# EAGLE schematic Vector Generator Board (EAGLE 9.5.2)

## Sheet 1 of 13: Power Supply & Negative Voltage generation
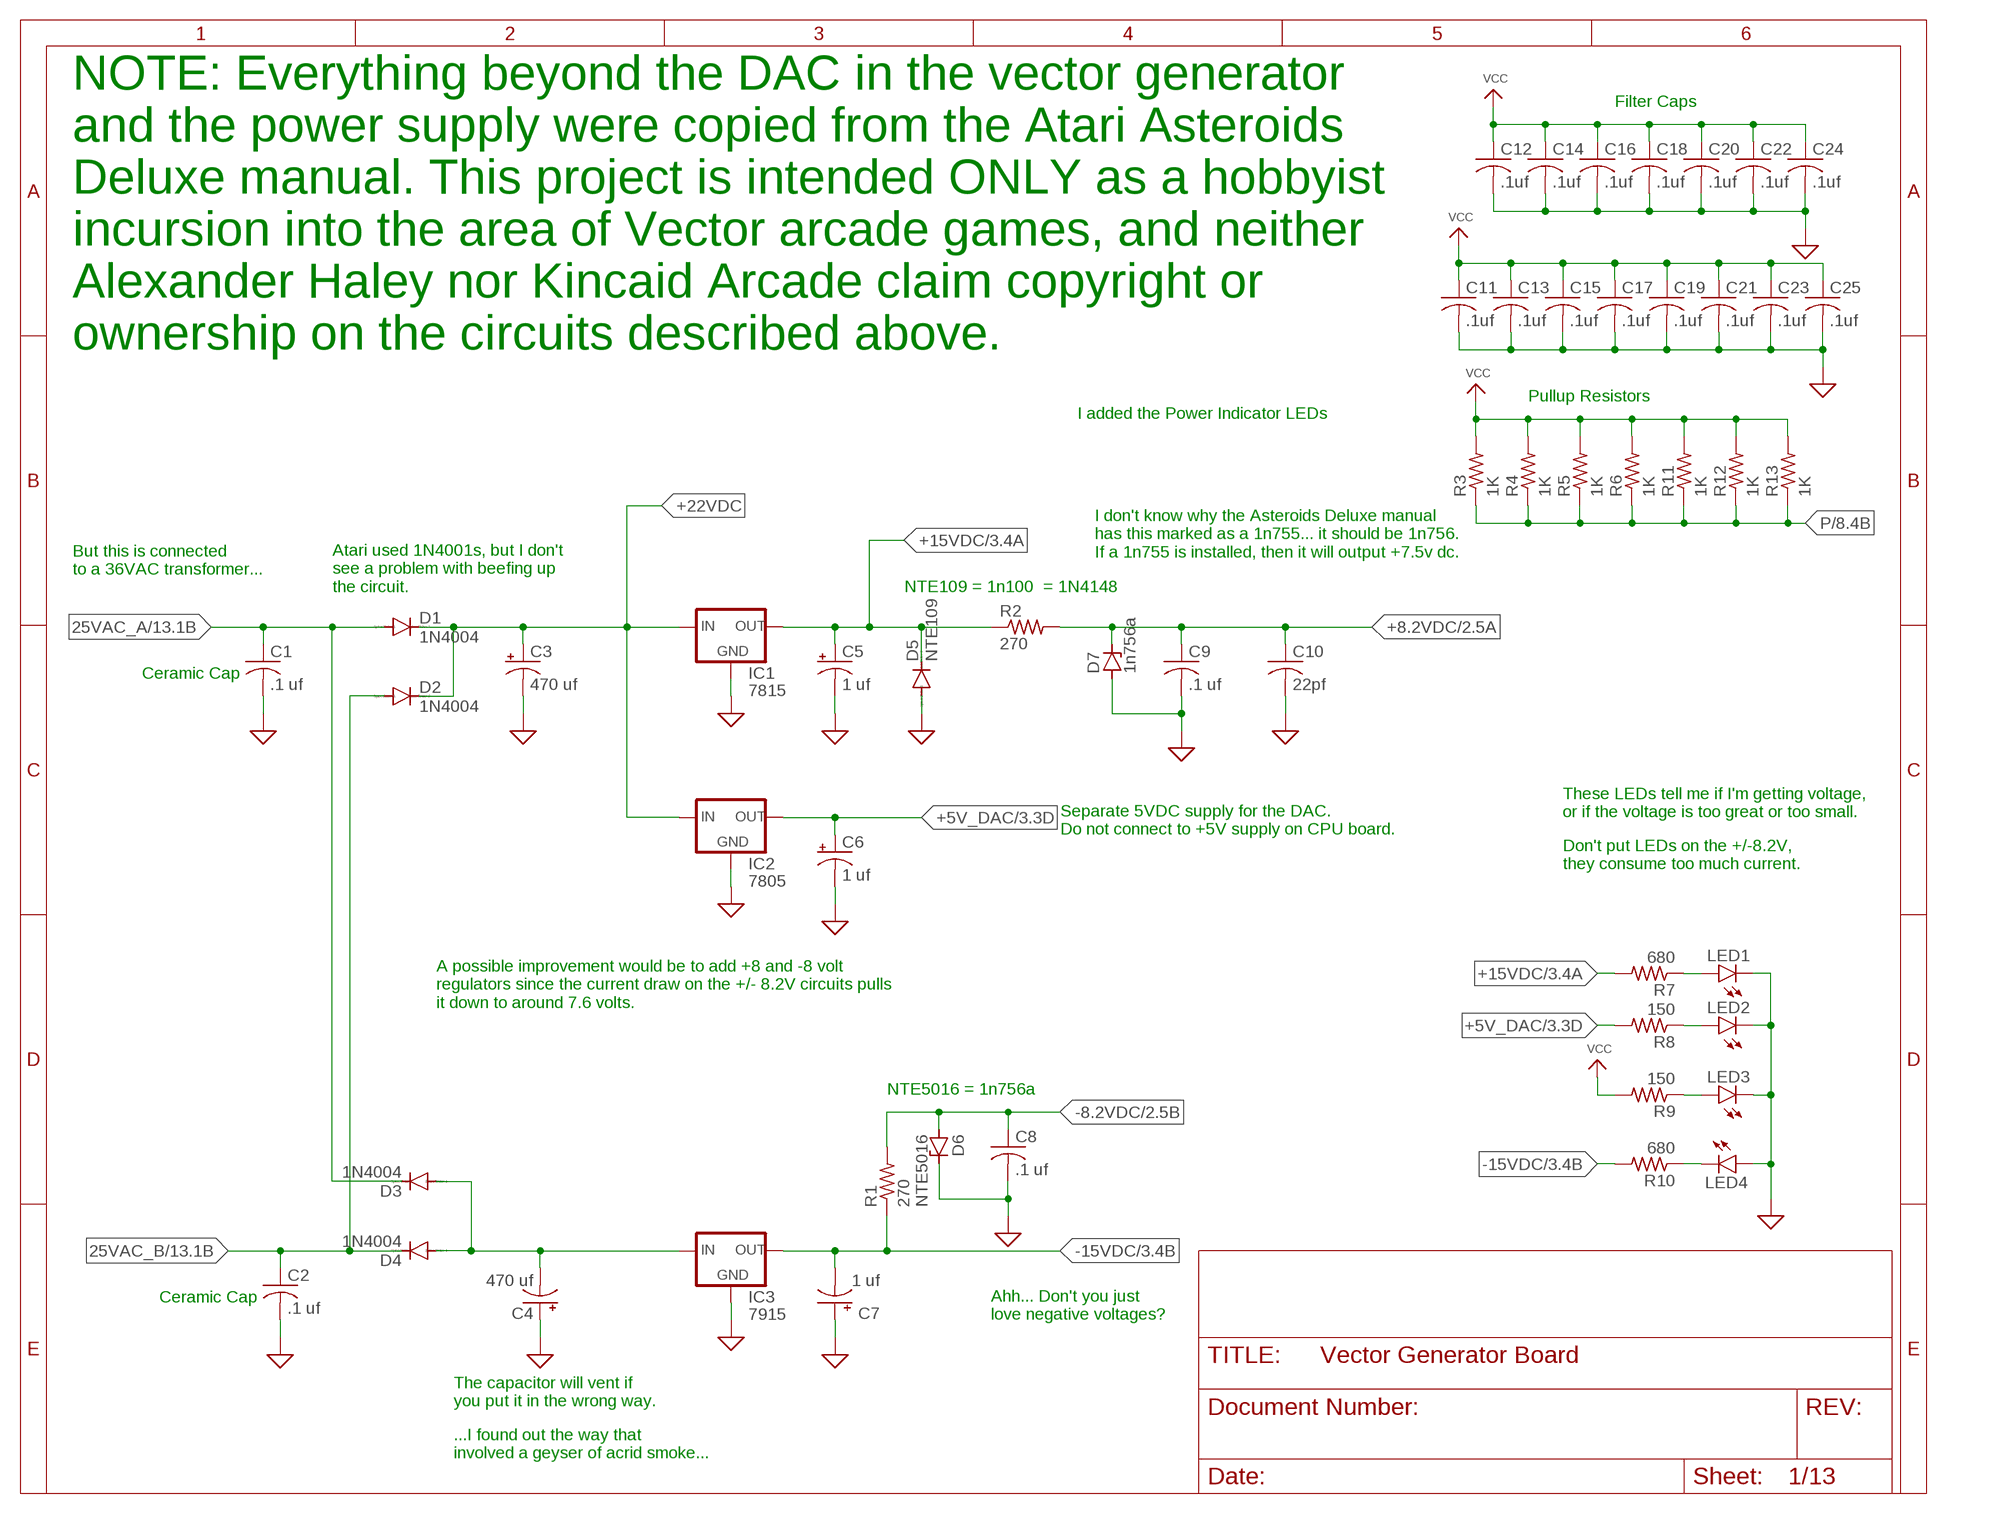
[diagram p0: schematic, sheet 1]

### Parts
C1  .1 uf  C-US050-050X075  [C050-050X075]
C2  .1 uf  C-US050-050X075  [C050-050X075]
C3  470 uf  CPOL-USE10-22.5  [EB22,5D]
C4  470 uf  CPOL-USE10-22.5  [EB22,5D]
C5  1 uf  CPOL-USB45181B  [B45181B]
C6  1 uf  CPOL-USB45181B  [B45181B]
C7  1 uf  CPOL-USB45181B  [B45181B]
C8  .1 uf  C-US050-050X075  [C050-050X075]
C9  .1 uf  C-US050-050X075  [C050-050X075]
C10  22pf  C-US050-050X075  [C050-050X075]
C11  .1uf  C-US050-030X075  [C050-030X075]
C12  .1uf  C-US050-030X075  [C050-030X075]
C13  .1uf  C-US050-030X075  [C050-030X075]
C14  .1uf  C-US050-030X075  [C050-030X075]
C15  .1uf  C-US050-030X075  [C050-030X075]
C16  .1uf  C-US050-030X075  [C050-030X075]
C17  .1uf  C-US050-030X075  [C050-030X075]
C18  .1uf  C-US050-030X075  [C050-030X075]
C19  .1uf  C-US050-030X075  [C050-030X075]
C20  .1uf  C-US050-030X075  [C050-030X075]
C21  .1uf  C-US050-030X075  [C050-030X075]
C22  .1uf  C-US050-030X075  [C050-030X075]
C23  .1uf  C-US050-030X075  [C050-030X075]
C24  .1uf  C-US050-030X075  [C050-030X075]
C25  .1uf  C-US050-030X075  [C050-030X075]
D1  1N4004  [DO41-10]
D2  1N4004  [DO41-10]
D3  1N4004  [DO41-10]
D4  1N4004  [DO41-10]
D5  NTE109  1N4004  [DO41-10]
D6  NTE5016  ZENER-DIODEDO35Z10  [DO35Z10]
D7  1n756a  ZENER-DIODEDO35Z10  [DO35Z10]
IC1  7815  78XXL  [78XXL]
IC2  7805  78XXL  [78XXL]
IC3  7915  78XXL  [78XXL]
LED1  LED3MM  [LED3MM]
LED2  LED3MM  [LED3MM]
LED3  LED3MM  [LED3MM]
LED4  LED3MM  [LED3MM]
R1  270  R-US_0207/12  [0207/12]
R2  270  R-US_0207/12  [0207/12]
R3  1K  R-US_0207/12  [0207/12]
R4  1K  R-US_0207/12  [0207/12]
R5  1K  R-US_0207/12  [0207/12]
R6  1K  R-US_0207/12  [0207/12]
R7  680  R-US_0207/12  [0207/12]
R8  150  R-US_0207/12  [0207/12]
R9  150  R-US_0207/12  [0207/12]
R10  680  R-US_0207/12  [0207/12]
R11  1K  R-US_0207/12  [0207/12]
R12  1K  R-US_0207/12  [0207/12]
R13  1K  R-US_0207/12  [0207/12]

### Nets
25VAC_A: C1.1 D1.A D3.C ; also sheet 13
25VAC_B: C2.1 D2.A D4.C ; also sheet 13
+5V_DAC: C6.+ IC2.OUT R8.2 ; also sheet 3,4
+8.2VDC: C9.1 C10.1 D7.C R2.2 ; also sheet 2,3,4,5
+15VDC: C5.+ D5.C IC1.OUT R2.1 R7.2 ; also sheet 3,4
+22VDC: C3.+ D1.C D2.C IC1.IN IC2.IN
-8.2VDC: C8.1 D6.A R1.2 ; also sheet 2,3,4,5
-15VDC: C7.- IC3.OUT R1.1 R10.2 ; also sheet 3,4
GND: C1.2 C2.2 C3.- C4.+ C5.- C6.- C7.+ C8.2 C9.2 C10.2 C11.2 C12.2 C13.2 C14.2 C15.2 C16.2 C17.2 C18.2 C19.2 C20.2 C21.2 C22.2 C23.2 C24.2 C25.2 D5.A D6.C D7.A IC1.GND IC2.GND IC3.GND LED1.K(C) LED2.K(C) LED3.K(C) LED4.A ; supply symbol labelled SUP ; also sheet 2,3,4,6,7,9,12,13
N$1: C4.- D3.A D4.A IC3.IN
N$6: LED1.A R7.1
N$8: LED2.A R8.1
N$9: LED3.A R9.1
N$123: LED4.K(C) R10.1
P: R3.1 R4.1 R5.1 R6.1 R11.1 R12.1 R13.1 ; also sheet 8,10,11,12
VCC: C11.1 C12.1 C13.1 C14.1 C15.1 C16.1 C17.1 C18.1 C19.1 C20.1 C21.1 C22.1 C23.1 C24.1 C25.1 R3.2 R4.2 R5.2 R6.2 R9.2 R11.2 R12.2 R13.2 ; also sheet 2,13

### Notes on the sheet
- Filter Caps
- NOTE: Everything beyond the DAC in the vector generator 
  and the power supply were copied from the Atari Asteroids 
  Deluxe manual. This project is intended ONLY as a hobbyist 
  incursion into the area of Vector arcade games, and neither 
  Alexander Haley nor Kincaid Arcade claim copyright or 
  ownership on the circuits described above.
- Pullup Resistors
- I added the Power Indicator LEDs
- I don't know why the Asteroids Deluxe manual
  has this marked as a 1n755... it should be 1n756.
  If a 1n755 is installed, then it will output +7.5v dc.
- But this is connected
  to a 36VAC transformer...
- Atari used 1N4001s, but I don't
  see a problem with beefing up
  the circuit.
- NTE109 = 1n100 | = 1N4148
- Ceramic Cap
- These LEDs tell me if I'm getting voltage,
  or if the voltage is too great or too small.
- Separate 5VDC supply for the DAC.
  Do not connect to +5V supply on CPU board.
- Don't put LEDs on the +/-8.2V,
  they consume too much current.
- A possible improvement would be to add +8 and -8 volt 
  regulators since the current draw on the +/- 8.2V circuits pulls 
  it down to around 7.6 volts.
- NTE5016 = 1n756a
- Ceramic Cap
- Ahh... Don't you just
  love negative voltages?
- The capacitor will vent if
  you put it in the wrong way.
- ...I found out the way that 
  involved a geyser of acrid smoke...

## Sheet 2 of 13: Z (Intensity) Out
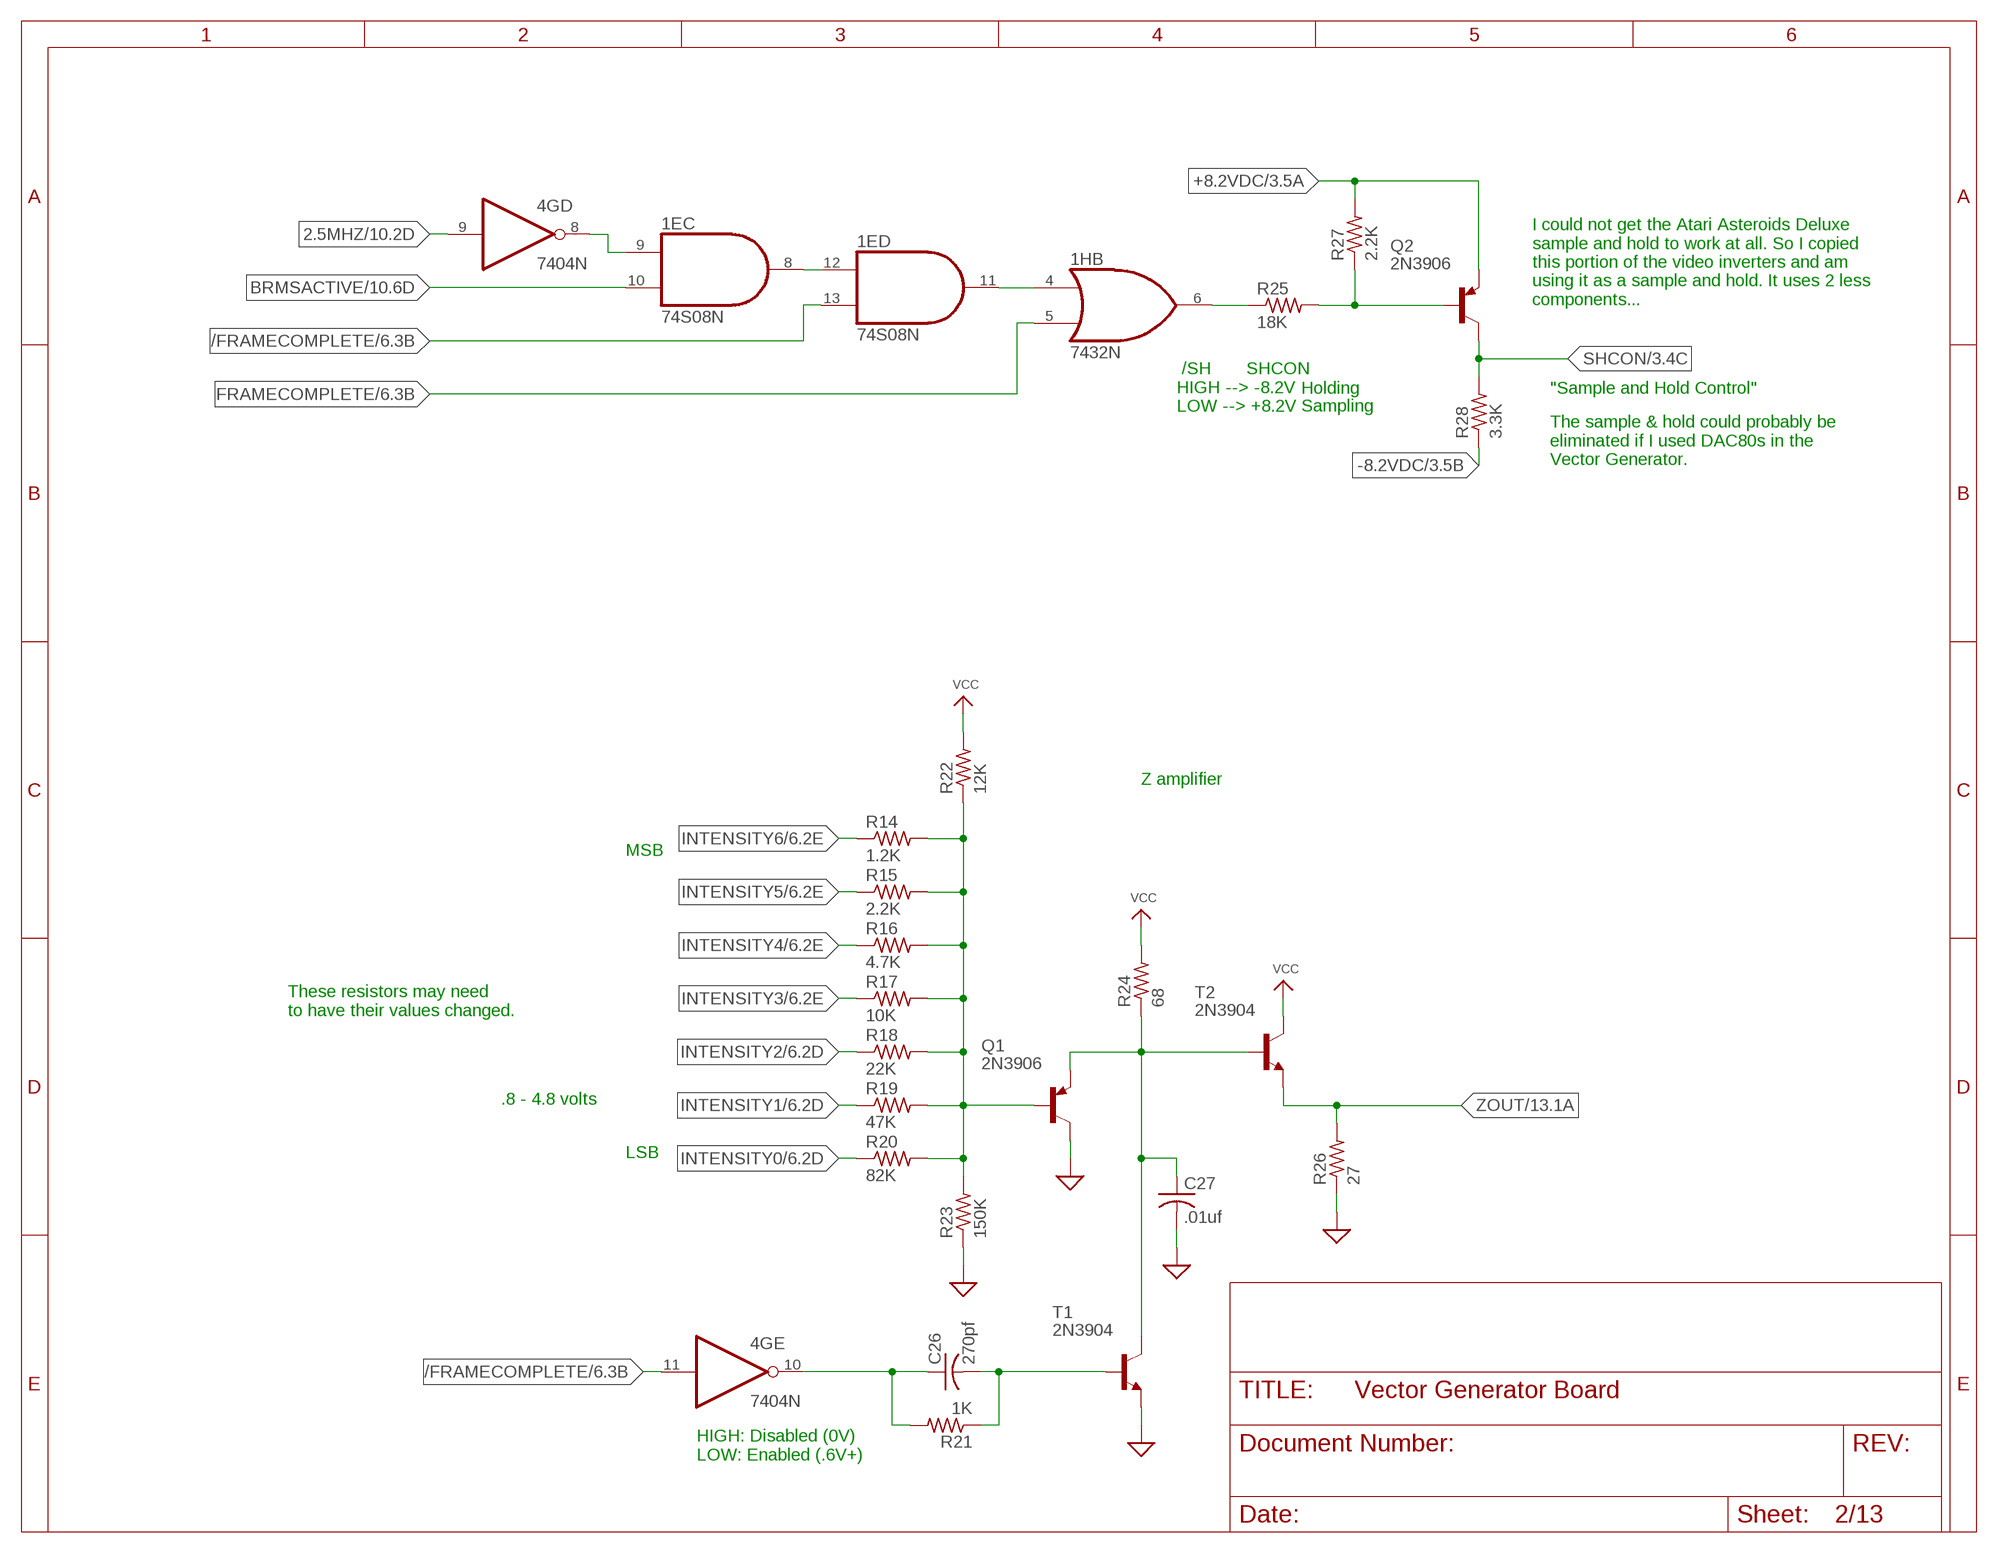
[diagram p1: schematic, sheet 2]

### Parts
1E  74S08N  [DIL14]
1H  7432N  [DIL14]
4G  7404N  [DIL14]
C26  270pf  C-US050-050X075  [C050-050X075]
C27  .01uf  C-US050-050X075  [C050-050X075]
Q1  2N3906  [TO92]
Q2  2N3906  [TO92]
R14  1.2K  R-US_0207/12  [0207/12]
R15  2.2K  R-US_0207/12  [0207/12]
R16  4.7K  R-US_0207/12  [0207/12]
R17  10K  R-US_0207/12  [0207/12]
R18  22K  R-US_0207/12  [0207/12]
R19  47K  R-US_0207/12  [0207/12]
R20  82K  R-US_0207/12  [0207/12]
R21  1K  R-US_0207/12  [0207/12]
R22  12K  R-US_0207/12  [0207/12]
R23  150K  R-US_0207/12  [0207/12]
R24  68  R-US_0207/12  [0207/12]
R25  18K  R-US_0207/12  [0207/12]
R26  27  R-US_0207/12  [0207/12]
R27  2.2K  R-US_0207/12  [0207/12]
R28  3.3K  R-US_0207/12  [0207/12]
T1  2N3904  [TO92]
T2  2N3904  [TO92]

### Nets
2.5MHZ: 4G.9(D:I) ; also sheet 10,13
+8.2VDC: Q2.3(E) R27.2 ; also sheet 1,3,4,5
-8.2VDC: R28.1 ; also sheet 1,3,4,5
/FRAMECOMPLETE: 1E.13(D:I1) 4G.11(E:I) ; also sheet 6
BRMSACTIVE: 1E.10(C:I1) ; also sheet 10
FRAMECOMPLETE: 1H.5(B:I1) ; also sheet 6,13
GND: C27.2 Q1.1(C) R23.1 R26.1 T1.3(E) ; supply symbol labelled SUP ; also sheet 1,3,4,6,7,9,12,13
INTENSITY0: R20.1 ; also sheet 6,11
INTENSITY1: R19.1 ; also sheet 6,11
INTENSITY2: R18.1 ; also sheet 6,11
INTENSITY3: R17.1 ; also sheet 6,11
INTENSITY4: R16.1 ; also sheet 6,11
INTENSITY5: R15.1 ; also sheet 6,11
INTENSITY6: R14.1 ; also sheet 6,11
N$2: 1H.6(B:O) R25.1
N$3: 1E.11(D:O) 1H.4(B:I0)
N$4: Q1.2(B) R14.2 R15.2 R16.2 R17.2 R18.2 R19.2 R20.2 R22.1 R23.2
N$5: Q2.2(B) R25.2 R27.1
N$12: C27.1 Q1.3(E) R24.1 T1.1(C) T2.2(B)
N$14: C26.2 R21.1 T1.2(B)
N$15: 4G.10(E:O) C26.1 R21.2
N$46: 1E.8(C:O) 1E.12(D:I0)
N$100: 1E.9(C:I0) 4G.8(D:O)
SHCON: Q2.1(C) R28.2 ; also sheet 3,4
VCC: R22.2 R24.2 T2.1(C) ; also sheet 1,13
ZOUT: R26.2 T2.3(E) ; also sheet 13

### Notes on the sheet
- I could not get the Atari Asteroids Deluxe
  sample and hold to work at all. So I copied
  this portion of the video inverters and am
  using it as a sample and hold. It uses 2 less
  components...
- Holding | "Sample and Hold Control"
- /SH       SHCON
  HIGH --> -8.2V
  LOW --> +8.2V
- Sampling
- The sample & hold could probably be 
  eliminated if I used DAC80s in the 
  Vector Generator.
- Z amplifier
- MSB
- These resistors may need 
  to have their values changed.
- .8 - 4.8 volts
- LSB
- HIGH: Disabled (0V)
  LOW: Enabled (.6V+)

## Sheet 3 of 13: X Out
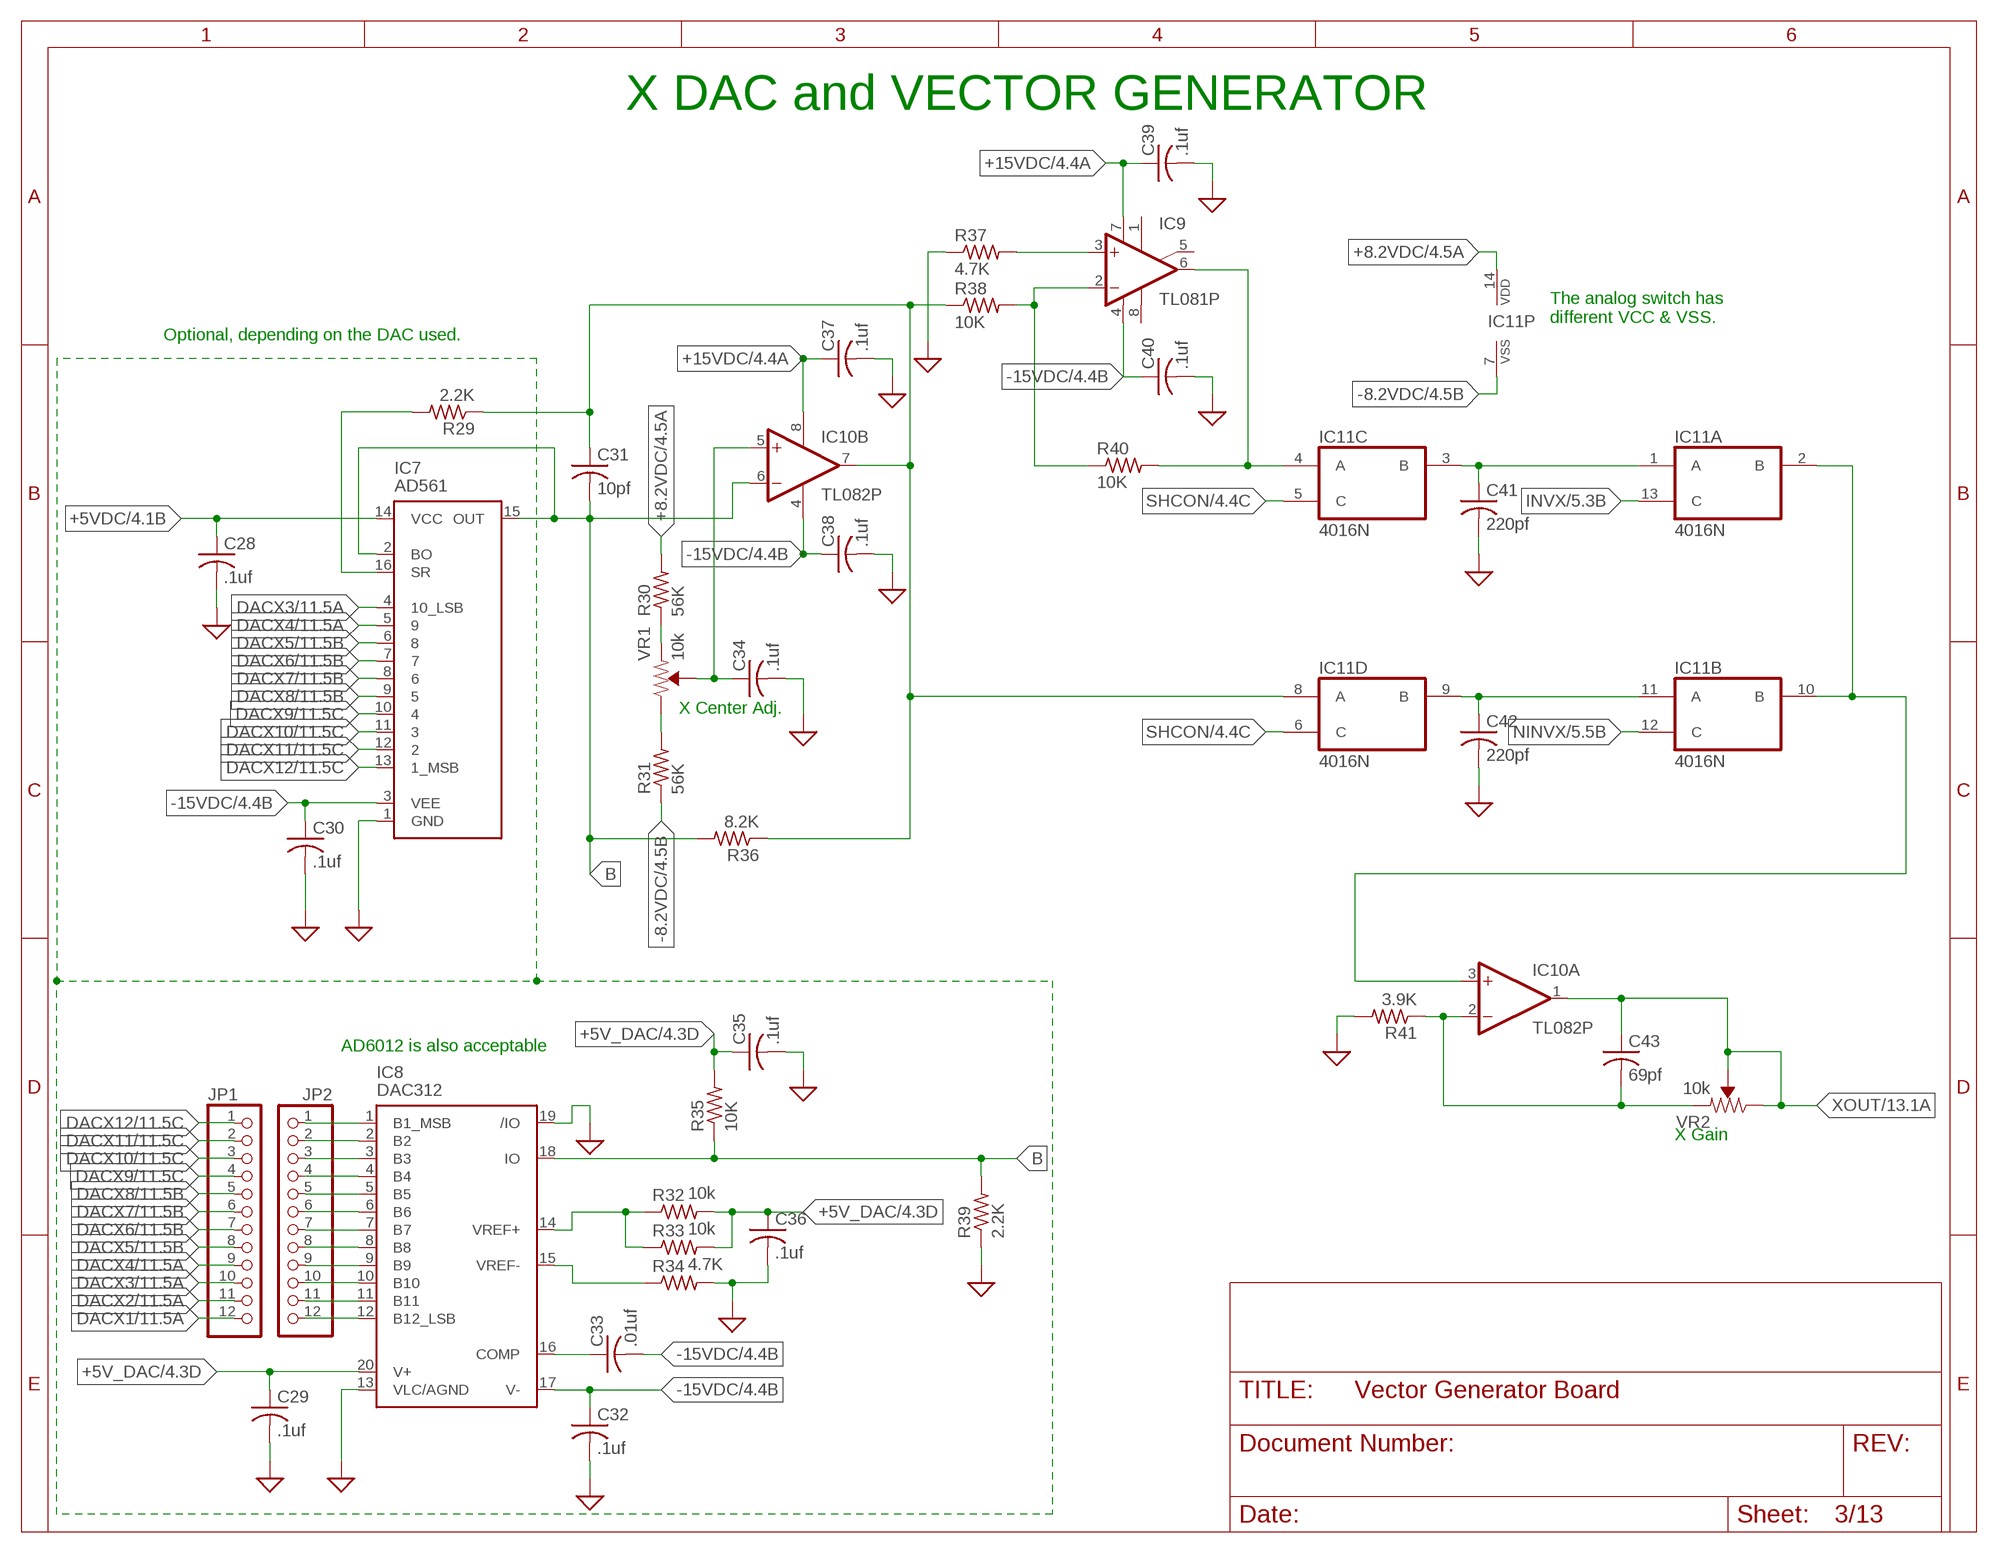
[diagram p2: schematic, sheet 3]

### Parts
C28  .1uf  C-US050-050X075  [C050-050X075]
C29  .1uf  C-US050-050X075  [C050-050X075]
C30  .1uf  C-US050-050X075  [C050-050X075]
C31  10pf  C-US050-050X075  [C050-050X075]
C32  .1uf  C-US050-050X075  [C050-050X075]
C33  .01uf  C-US050-050X075  [C050-050X075]
C34  .1uf  C-US050-050X075  [C050-050X075]
C35  .1uf  C-US050-050X075  [C050-050X075]
C36  .1uf  C-US050-050X075  [C050-050X075]
C37  .1uf  C-US050-050X075  [C050-050X075]
C38  .1uf  C-US050-050X075  [C050-050X075]
C39  .1uf  C-US050-050X075  [C050-050X075]
C40  .1uf  C-US050-050X075  [C050-050X075]
C41  220pf  C-US050-050X075  [C050-050X075]
C42  220pf  C-US050-050X075  [C050-050X075]
C43  69pf  C-US050-050X075  [C050-050X075]
IC7  AD561  [DIL16]
IC8  DAC312  [DIL20]
IC9  TL081P  [DIL08]
IC10  TL082P  [DIL08]
IC11  4016N  [DIL14]
JP1  PINHD-1X12  [1X12]
JP2  PINHD-1X12  [1X12]
R29  2.2K  R-US_0207/12  [0207/12]
R30  56K  R-US_0207/12  [0207/12]
R31  56K  R-US_0207/12  [0207/12]
R32  10k  R-US_0207/12  [0207/12]
R33  10k  R-US_0207/12  [0207/12]
R34  4.7K  R-US_0207/12  [0207/12]
R35  10K  R-US_0207/12  [0207/12]
R36  8.2K  R-US_0207/12  [0207/12]
R37  4.7K  R-US_0207/12  [0207/12]
R38  10K  R-US_0207/12  [0207/12]
R39  2.2K  R-US_0207/12  [0207/12]
R40  10K  R-US_0207/12  [0207/12]
R41  3.9K  R-US_0207/12  [0207/12]
VR1  10k  TRIMPOT-PTH-10MM-KNOB-1/2W-10%  [TRIMPOT-PTH-3386U]
VR2  10k  TRIMPOT-PTH-10MM-KNOB-1/2W-10%  [TRIMPOT-PTH-3386U]

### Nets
+5V_DAC: C29.1 C35.1 C36.1 IC8.20(V+) R32.2 R33.2 R35.2 ; also sheet 1,4
+5VDC: C28.1 IC7.14(VCC) ; also sheet 4
+8.2VDC: IC11.14(P:VDD) R30.2 ; also sheet 1,2,4,5
+15VDC: C37.1 C39.1 IC9.7(V+) IC10.8(P:V+) ; also sheet 1,4
-8.2VDC: IC11.7(P:VSS) R31.1 ; also sheet 1,2,4,5
-15VDC: C30.1 C32.1 C33.2 C38.1 C40.1 IC7.3(VEE) IC8.17(V-) IC9.4(V-) IC10.4(P:V-) ; also sheet 1,4
B: C31.2 IC7.2(BO) IC7.15(OUT) IC8.18(IO) IC10.6(B:-IN) R35.1 R36.2 R39.2
DACX1: JP1.12 ; also sheet 11,12
DACX2: JP1.11 ; also sheet 11,12
DACX3: IC7.4(10_LSB) JP1.10 ; also sheet 11,12
DACX4: IC7.5 JP1.9 ; also sheet 11,12
DACX5: IC7.6 JP1.8 ; also sheet 11,12
DACX6: IC7.7 JP1.7 ; also sheet 11,12
DACX7: IC7.8 JP1.6 ; also sheet 11,12
DACX8: IC7.9 JP1.5 ; also sheet 11,12
DACX9: IC7.10 JP1.4 ; also sheet 11,12
DACX10: IC7.11 JP1.3 ; also sheet 11,12
DACX11: IC7.12 JP1.2 ; also sheet 11,12
DACX12: IC7.13(1_MSB) JP1.1 ; also sheet 11,12
GND: C28.2 C29.2 C30.2 C32.2 C34.2 C35.2 C36.2 C37.2 C38.2 C39.2 C40.2 C41.2 C42.2 IC7.1(GND) IC8.13(VLC/AGND) IC8.19(/IO) R34.2 R37.1 R39.1 R41.2 ; supply symbol labelled SUP ; also sheet 1,2,4,6,7,9,12,13
INVX: IC11.13(A:C) ; also sheet 5
N$11: C31.1 IC10.7(B:OUT) IC11.8(D:A) R29.1 R36.1 R38.1
N$13: IC7.16(SR) R29.2
N$16: C41.1 IC11.1(A:A) IC11.3(C:B)
N$17: C42.1 IC11.9(D:B) IC11.11(B:A)
N$18: IC10.3(A:+IN) IC11.2(A:B) IC11.10(B:B)
N$19: IC9.2(-IN) R38.2 R40.1
N$20: IC9.3(+IN) R37.2
N$21: IC9.6(OUT) IC11.4(C:A) R40.2
N$23: C43.2 IC10.2(A:-IN) R41.1 VR2.1(CCW)
N$57: R31.2 VR1.3(CW)
N$108: IC8.1(B1_MSB) JP2.1
N$109: IC8.2(B2) JP2.2
N$110: IC8.3(B3) JP2.3
N$119: R30.1 VR1.1(CCW)
N$120: C33.1 IC8.16(COMP)
N$121: IC8.14(VREF+) R32.1 R33.1
N$122: IC8.15(VREF-) R34.1
N$124: C34.1 IC10.5(B:+IN) VR1.2(WIPER)
N$125: IC8.4(B4) JP2.4
N$128: IC8.5(B5) JP2.5
N$130: IC8.6(B6) JP2.6
N$131: IC8.7(B7) JP2.7
N$132: IC8.8(B8) JP2.8
N$133: IC8.9(B9) JP2.9
N$134: IC8.10(B10) JP2.10
N$135: IC8.11(B11) JP2.11
N$136: IC8.12(B12_LSB) JP2.12
NINVX: IC11.12(B:C) ; also sheet 5
SHCON: IC11.5(C:C) IC11.6(D:C) ; also sheet 2,4
XOUT: C43.1 IC10.1(A:OUT) VR2.2(WIPER) VR2.3(CW) ; also sheet 13
Unconnected: IC9.1(ON1) IC9.5(ON2) IC9.8(OPT)

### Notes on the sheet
- X DAC and VECTOR GENERATOR
- The analog switch has
  different VCC & VSS.
- Optional, depending on the DAC used.
- X Center Adj.
- AD6012 is also acceptable
- X Gain

## Sheet 4 of 13: Y Out
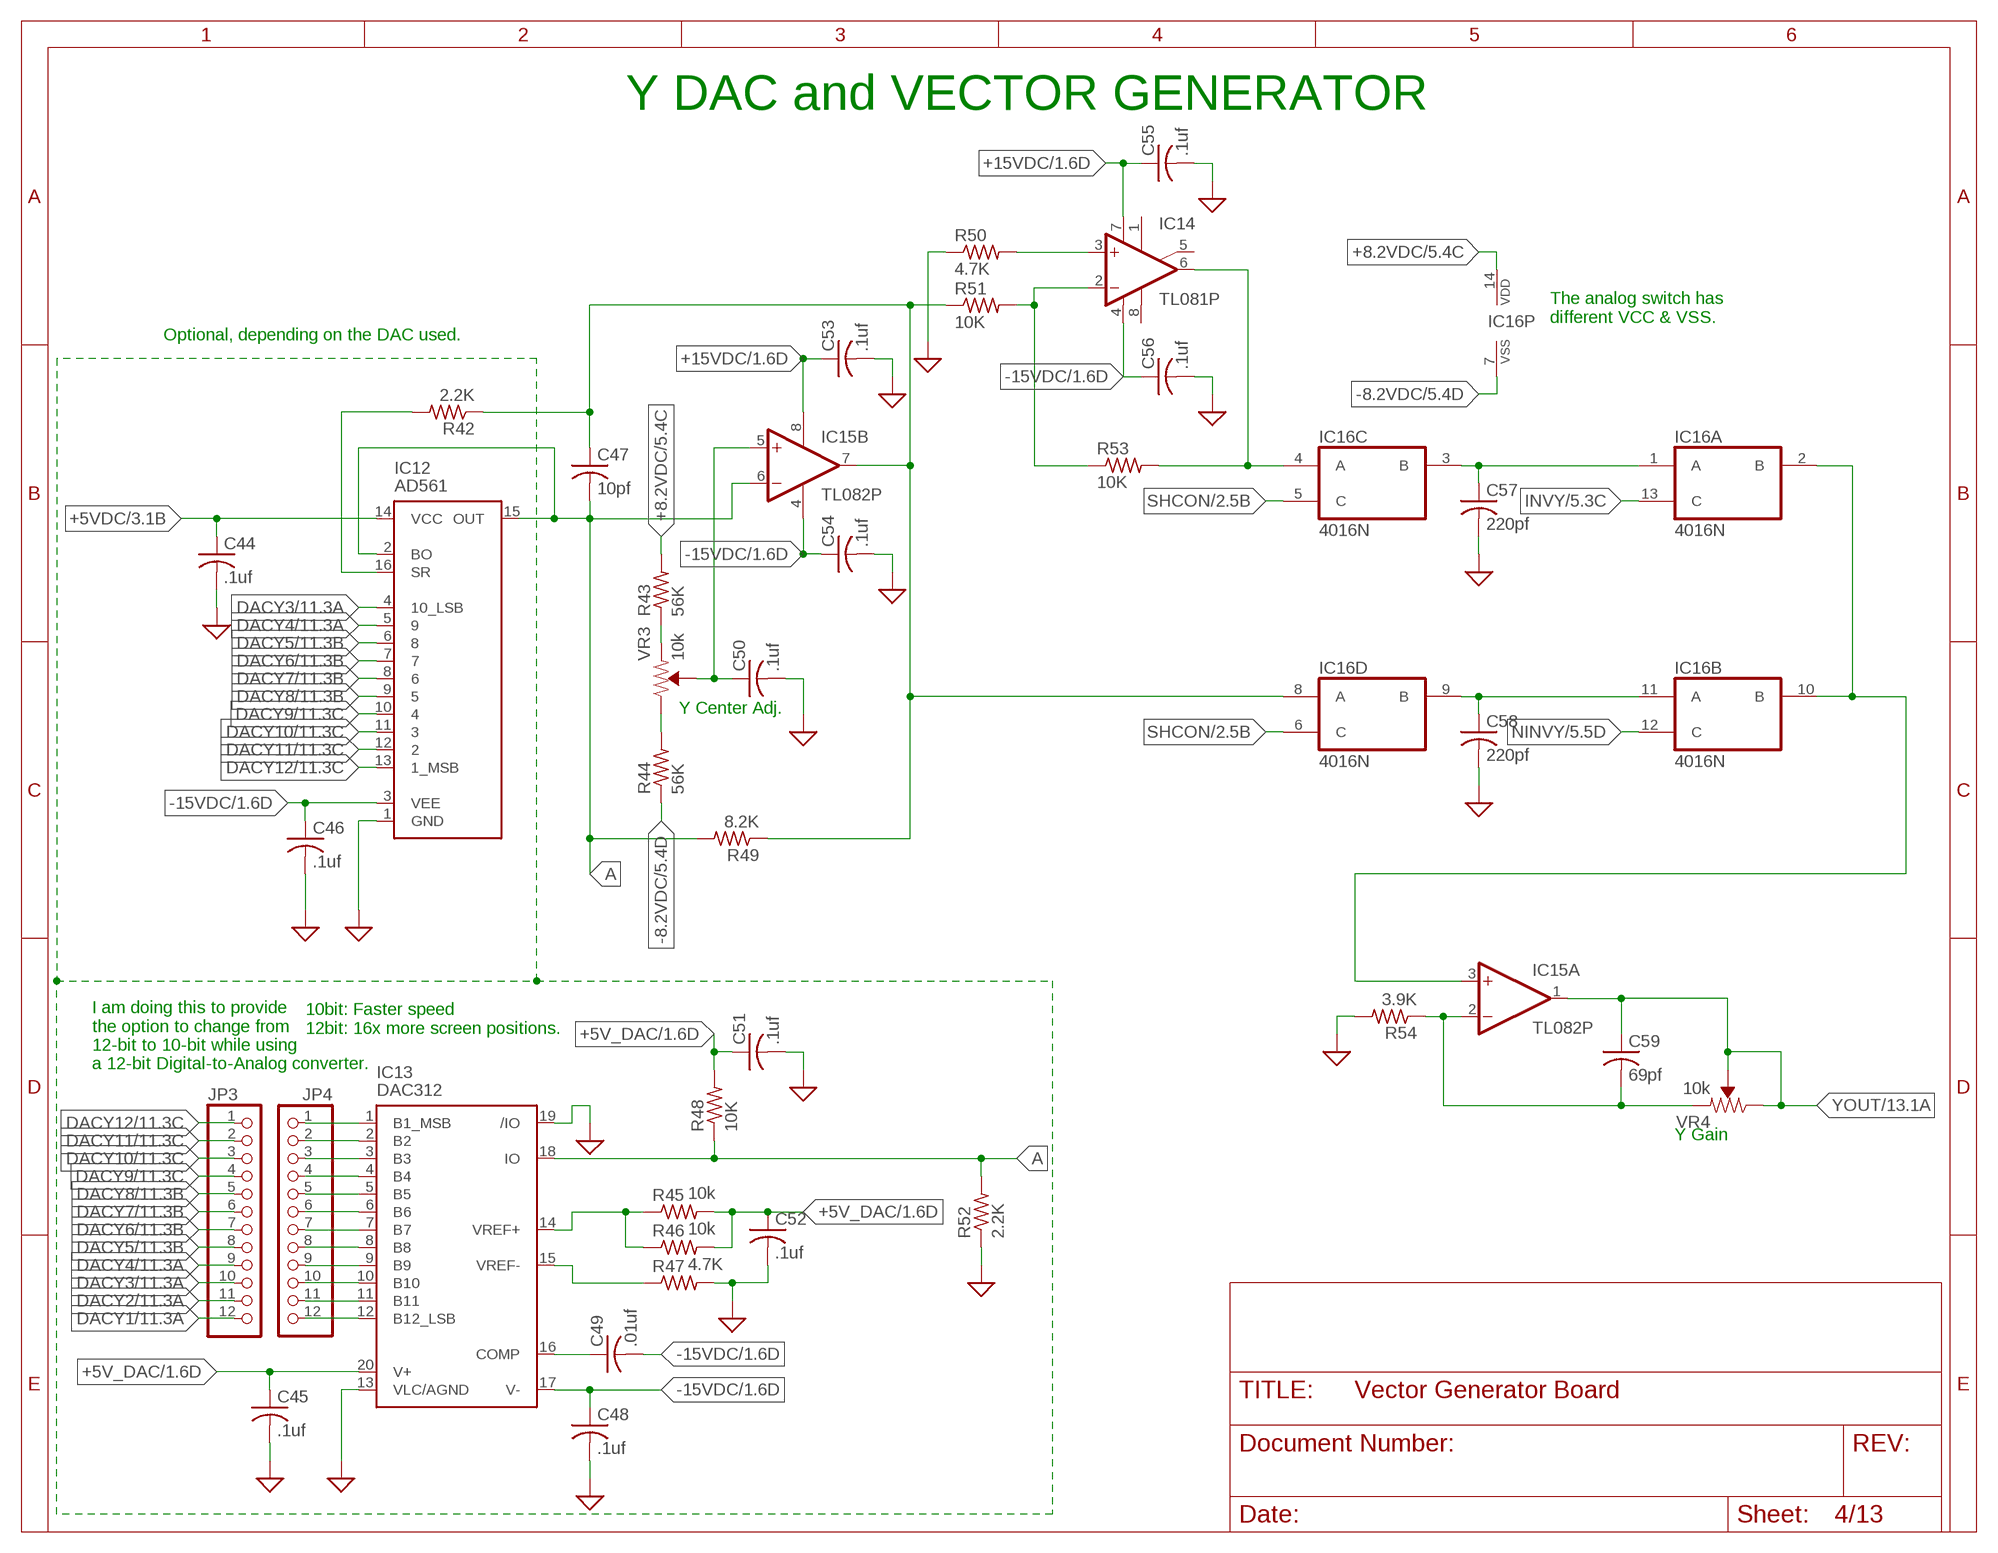
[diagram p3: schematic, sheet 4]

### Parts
C44  .1uf  C-US050-050X075  [C050-050X075]
C45  .1uf  C-US050-050X075  [C050-050X075]
C46  .1uf  C-US050-050X075  [C050-050X075]
C47  10pf  C-US050-050X075  [C050-050X075]
C48  .1uf  C-US050-050X075  [C050-050X075]
C49  .01uf  C-US050-050X075  [C050-050X075]
C50  .1uf  C-US050-050X075  [C050-050X075]
C51  .1uf  C-US050-050X075  [C050-050X075]
C52  .1uf  C-US050-050X075  [C050-050X075]
C53  .1uf  C-US050-050X075  [C050-050X075]
C54  .1uf  C-US050-050X075  [C050-050X075]
C55  .1uf  C-US050-050X075  [C050-050X075]
C56  .1uf  C-US050-050X075  [C050-050X075]
C57  220pf  C-US050-050X075  [C050-050X075]
C58  220pf  C-US050-050X075  [C050-050X075]
C59  69pf  C-US050-050X075  [C050-050X075]
IC12  AD561  [DIL16]
IC13  DAC312  [DIL20]
IC14  TL081P  [DIL08]
IC15  TL082P  [DIL08]
IC16  4016N  [DIL14]
JP3  PINHD-1X12  [1X12]
JP4  PINHD-1X12  [1X12]
R42  2.2K  R-US_0207/12  [0207/12]
R43  56K  R-US_0207/12  [0207/12]
R44  56K  R-US_0207/12  [0207/12]
R45  10k  R-US_0207/12  [0207/12]
R46  10k  R-US_0207/12  [0207/12]
R47  4.7K  R-US_0207/12  [0207/12]
R48  10K  R-US_0207/12  [0207/12]
R49  8.2K  R-US_0207/12  [0207/12]
R50  4.7K  R-US_0207/12  [0207/12]
R51  10K  R-US_0207/12  [0207/12]
R52  2.2K  R-US_0207/12  [0207/12]
R53  10K  R-US_0207/12  [0207/12]
R54  3.9K  R-US_0207/12  [0207/12]
VR3  10k  TRIMPOT-PTH-10MM-KNOB-1/2W-10%  [TRIMPOT-PTH-3386U]
VR4  10k  TRIMPOT-PTH-10MM-KNOB-1/2W-10%  [TRIMPOT-PTH-3386U]

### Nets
+5V_DAC: C45.1 C51.1 C52.1 IC13.20(V+) R45.2 R46.2 R48.2 ; also sheet 1,3
+5VDC: C44.1 IC12.14(VCC) ; also sheet 3
+8.2VDC: IC16.14(P:VDD) R43.2 ; also sheet 1,2,3,5
+15VDC: C53.1 C55.1 IC14.7(V+) IC15.8(P:V+) ; also sheet 1,3
-8.2VDC: IC16.7(P:VSS) R44.1 ; also sheet 1,2,3,5
-15VDC: C46.1 C48.1 C49.2 C54.1 C56.1 IC12.3(VEE) IC13.17(V-) IC14.4(V-) IC15.4(P:V-) ; also sheet 1,3
A: C47.2 IC12.2(BO) IC12.15(OUT) IC13.18(IO) IC15.6(B:-IN) R48.1 R49.2 R52.2
DACY1: JP3.12 ; also sheet 11,12
DACY2: JP3.11 ; also sheet 11,12
DACY3: IC12.4(10_LSB) JP3.10 ; also sheet 11,12
DACY4: IC12.5 JP3.9 ; also sheet 11,12
DACY5: IC12.6 JP3.8 ; also sheet 11,12
DACY6: IC12.7 JP3.7 ; also sheet 11,12
DACY7: IC12.8 JP3.6 ; also sheet 11,12
DACY8: IC12.9 JP3.5 ; also sheet 11,12
DACY9: IC12.10 JP3.4 ; also sheet 11,12
DACY10: IC12.11 JP3.3 ; also sheet 11,12
DACY11: IC12.12 JP3.2 ; also sheet 11,12
DACY12: IC12.13(1_MSB) JP3.1 ; also sheet 11,12
GND: C44.2 C45.2 C46.2 C48.2 C50.2 C51.2 C52.2 C53.2 C54.2 C55.2 C56.2 C57.2 C58.2 IC12.1(GND) IC13.13(VLC/AGND) IC13.19(/IO) R47.2 R50.1 R52.1 R54.2 ; supply symbol labelled SUP ; also sheet 1,2,3,6,7,9,12,13
INVY: IC16.13(A:C) ; also sheet 5
N$10: R44.2 VR3.3(CW)
N$22: IC13.1(B1_MSB) JP4.1
N$24: IC13.2(B2) JP4.2
N$25: C47.1 IC15.7(B:OUT) IC16.8(D:A) R42.1 R49.1 R51.1
N$26: IC12.16(SR) R42.2
N$27: C57.1 IC16.1(A:A) IC16.3(C:B)
N$28: C58.1 IC16.9(D:B) IC16.11(B:A)
N$29: IC15.3(A:+IN) IC16.2(A:B) IC16.10(B:B)
N$30: IC14.2(-IN) R51.2 R53.1
N$31: IC14.3(+IN) R50.2
N$32: IC14.6(OUT) IC16.4(C:A) R53.2
N$33: C59.2 IC15.2(A:-IN) R54.1 VR4.1(CCW)
N$44: IC13.3(B3) JP4.3
N$45: IC13.4(B4) JP4.4
N$54: IC13.5(B5) JP4.5
N$55: IC13.6(B6) JP4.6
N$56: IC13.7(B7) JP4.7
N$71: IC13.8(B8) JP4.8
N$98: IC13.9(B9) JP4.9
N$105: IC13.10(B10) JP4.10
N$106: IC13.11(B11) JP4.11
N$107: IC13.12(B12_LSB) JP4.12
N$115: IC13.14(VREF+) R45.1 R46.1
N$116: C49.1 IC13.16(COMP)
N$118: IC13.15(VREF-) R47.1
N$126: R43.1 VR3.1(CCW)
N$127: C50.1 IC15.5(B:+IN) VR3.2(WIPER)
NINVY: IC16.12(B:C) ; also sheet 5
SHCON: IC16.5(C:C) IC16.6(D:C) ; also sheet 2,3
YOUT: C59.1 IC15.1(A:OUT) VR4.2(WIPER) VR4.3(CW) ; also sheet 13
Unconnected: IC14.1(ON1) IC14.5(ON2) IC14.8(OPT)

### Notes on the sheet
- Y DAC and VECTOR GENERATOR
- The analog switch has
  different VCC & VSS.
- Optional, depending on the DAC used.
- Y Center Adj.
- 10bit: Faster speed
  12bit: 16x more screen positions.
- I am doing this to provide
  the option to change from
  12-bit to 10-bit while using
  a 12-bit Digital-to-Analog converter.
- Y Gain

## Sheet 5 of 13: Video Inverter
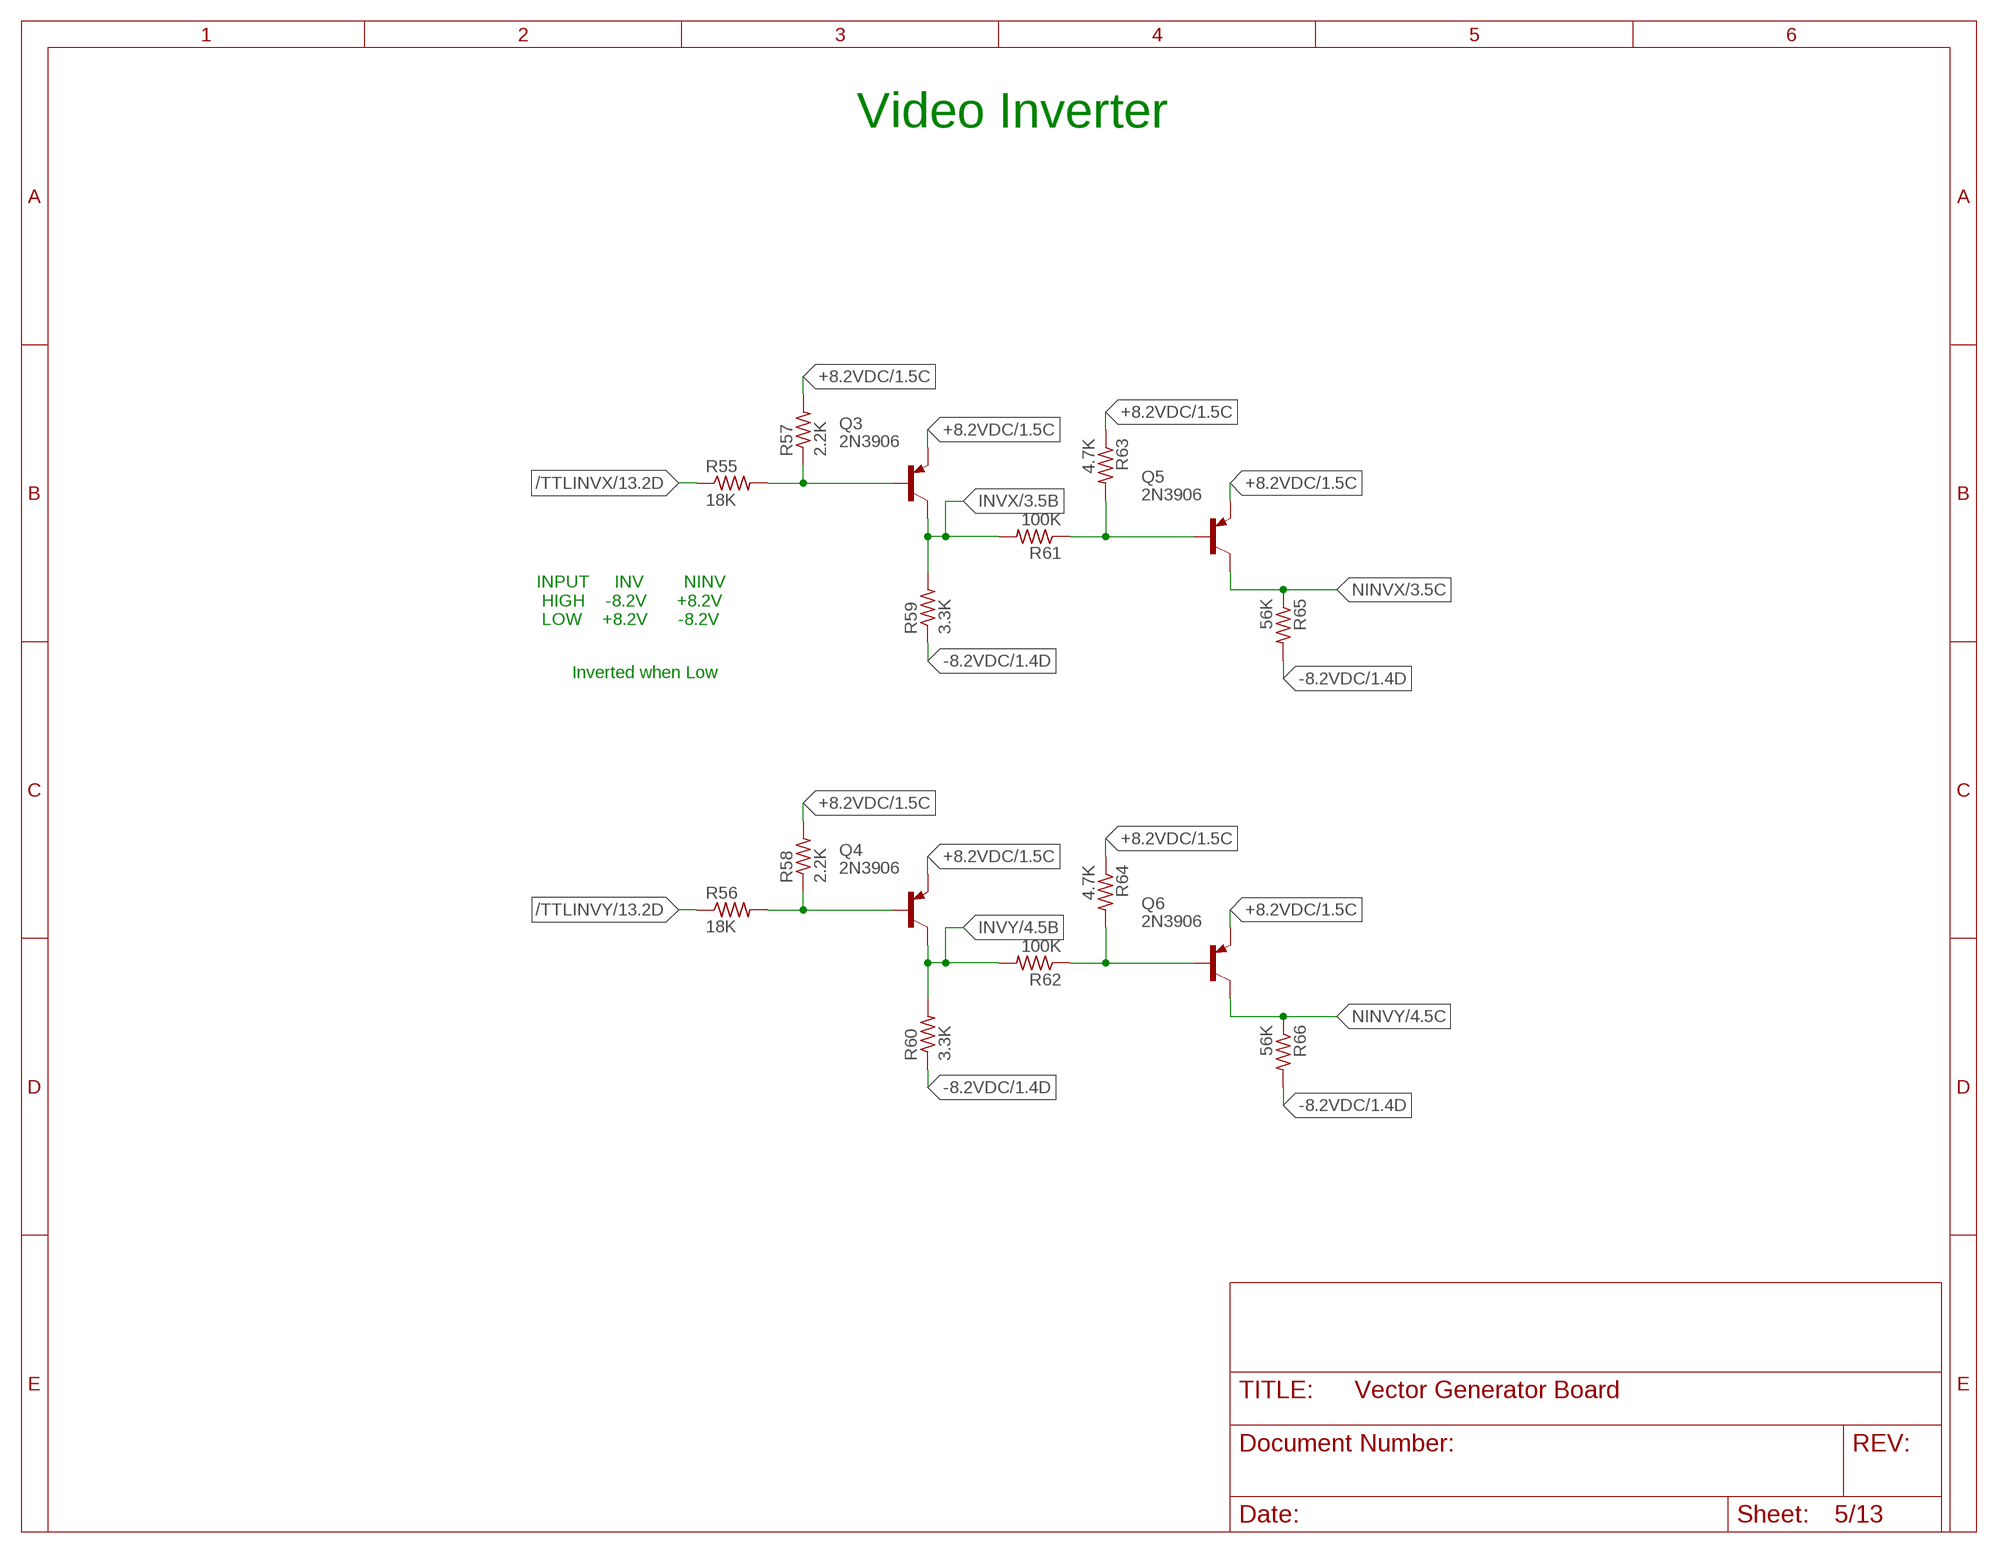
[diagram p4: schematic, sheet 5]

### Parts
Q3  2N3906  [TO92]
Q4  2N3906  [TO92]
Q5  2N3906  [TO92]
Q6  2N3906  [TO92]
R55  18K  R-US_0207/12  [0207/12]
R56  18K  R-US_0207/12  [0207/12]
R57  2.2K  R-US_0207/12  [0207/12]
R58  2.2K  R-US_0207/12  [0207/12]
R59  3.3K  R-US_0207/12  [0207/12]
R60  3.3K  R-US_0207/12  [0207/12]
R61  100K  R-US_0207/12  [0207/12]
R62  100K  R-US_0207/12  [0207/12]
R63  4.7K  R-US_0207/12  [0207/12]
R64  4.7K  R-US_0207/12  [0207/12]
R65  56K  R-US_0207/12  [0207/12]
R66  56K  R-US_0207/12  [0207/12]

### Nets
+8.2VDC: Q3.3(E) Q4.3(E) Q5.3(E) Q6.3(E) R57.2 R58.2 R63.1 R64.1 ; also sheet 1,2,3,4
-8.2VDC: R59.1 R60.1 R65.2 R66.2 ; also sheet 1,2,3,4
/TTLINVX: R55.1 ; also sheet 13
/TTLINVY: R56.1 ; also sheet 13
INVX: Q3.1(C) R59.2 R61.2 ; also sheet 3
INVY: Q4.1(C) R60.2 R62.2 ; also sheet 4
N$35: Q3.2(B) R55.2 R57.1
N$37: Q4.2(B) R56.2 R58.1
N$38: Q6.2(B) R62.1 R64.2
N$39: Q5.2(B) R61.1 R63.2
NINVX: Q5.1(C) R65.1 ; also sheet 3
NINVY: Q6.1(C) R66.1 ; also sheet 4

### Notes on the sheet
- Video Inverter
- INPUT     INV        NINV
   HIGH    -8.2V      +8.2V
   LOW    +8.2V      -8.2V
- Inverted when Low

## Sheet 6 of 13: Input Latches & Stage Counter
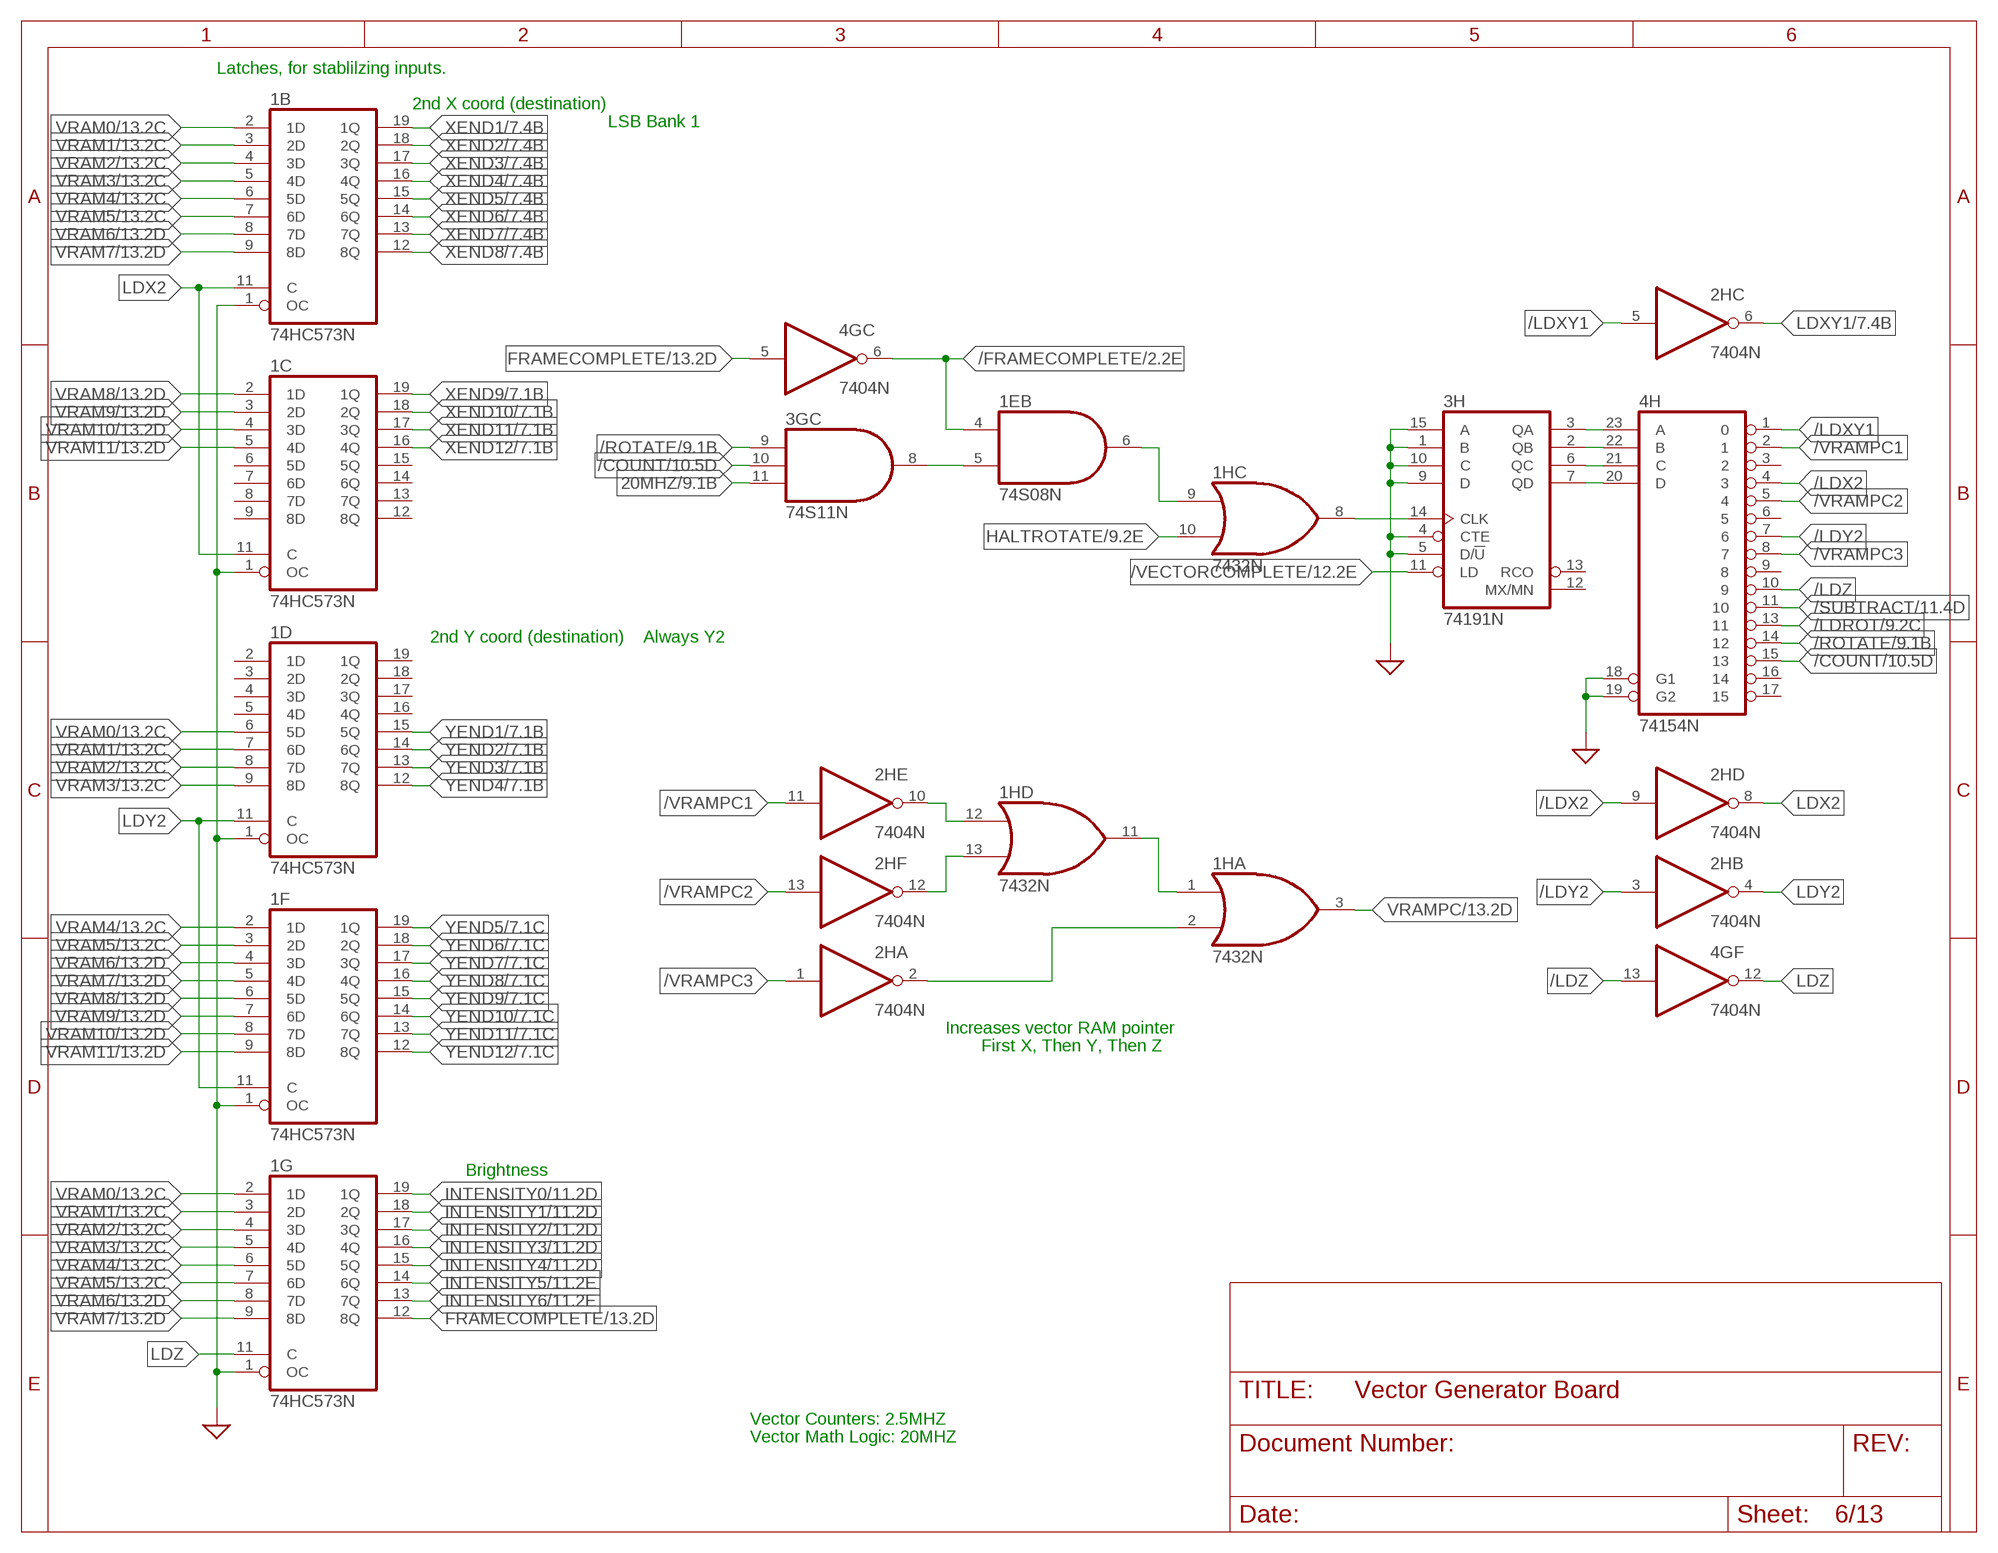
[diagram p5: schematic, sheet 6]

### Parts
1B  74HC573N  [DIL20]
1C  74HC573N  [DIL20]
1D  74HC573N  [DIL20]
1F  74HC573N  [DIL20]
1G  74HC573N  [DIL20]
2H  7404N  [DIL14]
3G  74S11N  [DIL14]
3H  74191N  [DIL16]
4H  74154N  [DIL24-6]

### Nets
20MHZ: 3G.11(C:I2) ; also sheet 9,13
/COUNT: 3G.10(C:I1) 4H.15 ; also sheet 10
/FRAMECOMPLETE: 1E.4(B:I0) 4G.6(C:O) ; also sheet 2
/LDROT: 4H.13 ; also sheet 9
/LDX2: 2H.9(D:I) 4H.4
/LDXY1: 2H.5(C:I) 4H.1
/LDY2: 2H.3(B:I) 4H.7
/LDZ: 4G.13(F:I) 4H.10
/ROTATE: 3G.9(C:I0) 4H.14 ; also sheet 9
/SUBTRACT: 4H.11 ; also sheet 11
/VECTORCOMPLETE: 3H.11(LD) ; also sheet 12
/VRAMPC1: 2H.11(E:I) 4H.2
/VRAMPC2: 2H.13(F:I) 4H.5
/VRAMPC3: 2H.1(A:I) 4H.8
FRAMECOMPLETE: 1G.12(8Q) 4G.5(C:I) ; also sheet 2,13
GND: 1B.1(OC) 1C.1(OC) 1D.1(OC) 1F.1(OC) 1G.1(OC) 3H.1(B) 3H.4(CTE) 3H.5(D/!U) 3H.9(D) 3H.10(C) 3H.15(A) 4H.18(G1) 4H.19(G2) ; supply symbol labelled SUP ; also sheet 1,2,3,4,7,9,12,13
HALTROTATE: 1H.10(C:I1) ; also sheet 9
INTENSITY0: 1G.19(1Q) ; also sheet 2,11
INTENSITY1: 1G.18(2Q) ; also sheet 2,11
INTENSITY2: 1G.17(3Q) ; also sheet 2,11
INTENSITY3: 1G.16(4Q) ; also sheet 2,11
INTENSITY4: 1G.15(5Q) ; also sheet 2,11
INTENSITY5: 1G.14(6Q) ; also sheet 2,11
INTENSITY6: 1G.13(7Q) ; also sheet 2,11
LDX2: 1B.11(C) 1C.11(C) 2H.8(D:O)
LDXY1: 2H.6(C:O) ; also sheet 7
LDY2: 1D.11(C) 1F.11(C) 2H.4(B:O)
LDZ: 1G.11(C) 4G.12(F:O)
N$48: 3H.3(QA) 4H.23(A)
N$49: 1H.8(C:O) 3H.14(CLK)
N$50: 3H.2(QB) 4H.22(B)
N$51: 3H.6(QC) 4H.21(C)
N$52: 3H.7(QD) 4H.20(D)
N$53: 1E.6(B:O) 1H.9(C:I0)
N$97: 1E.5(B:I1) 3G.8(C:O)
N$111: 1H.12(D:I0) 2H.10(E:O)
N$112: 1H.13(D:I1) 2H.12(F:O)
N$113: 1H.2(A:I1) 2H.2(A:O)
N$114: 1H.1(A:I0) 1H.11(D:O)
VRAM0: 1B.2(1D) 1D.6(5D) 1G.2(1D) ; also sheet 13
VRAM1: 1B.3(2D) 1D.7(6D) 1G.3(2D) ; also sheet 13
VRAM2: 1B.4(3D) 1D.8(7D) 1G.4(3D) ; also sheet 13
VRAM3: 1B.5(4D) 1D.9(8D) 1G.5(4D) ; also sheet 13
VRAM4: 1B.6(5D) 1F.2(1D) 1G.6(5D) ; also sheet 13
VRAM5: 1B.7(6D) 1F.3(2D) 1G.7(6D) ; also sheet 13
VRAM6: 1B.8(7D) 1F.4(3D) 1G.8(7D) ; also sheet 13
VRAM7: 1B.9(8D) 1F.5(4D) 1G.9(8D) ; also sheet 13
VRAM8: 1C.2(1D) 1F.6(5D) ; also sheet 13
VRAM9: 1C.3(2D) 1F.7(6D) ; also sheet 13
VRAM10: 1C.4(3D) 1F.8(7D) ; also sheet 13
VRAM11: 1C.5(4D) 1F.9(8D) ; also sheet 13
VRAMPC: 1H.3(A:O) ; also sheet 13
XEND1: 1B.19(1Q) ; also sheet 7,8,11,12
XEND2: 1B.18(2Q) ; also sheet 7,8,11,12
XEND3: 1B.17(3Q) ; also sheet 7,8,11,12
XEND4: 1B.16(4Q) ; also sheet 7,8,11,12
XEND5: 1B.15(5Q) ; also sheet 7,8,11,12
XEND6: 1B.14(6Q) ; also sheet 7,8,11,12
XEND7: 1B.13(7Q) ; also sheet 7,8,11,12
XEND8: 1B.12(8Q) ; also sheet 7,8,11,12
XEND9: 1C.19(1Q) ; also sheet 7,8,11,12
XEND10: 1C.18(2Q) ; also sheet 7,8,11,12
XEND11: 1C.17(3Q) ; also sheet 7,8,11,12
XEND12: 1C.16(4Q) ; also sheet 7,8,11,12
YEND1: 1D.15(5Q) ; also sheet 7,8,11,12
YEND2: 1D.14(6Q) ; also sheet 7,8,11,12
YEND3: 1D.13(7Q) ; also sheet 7,8,11,12
YEND4: 1D.12(8Q) ; also sheet 7,8,11,12
YEND5: 1F.19(1Q) ; also sheet 7,8,11,12
YEND6: 1F.18(2Q) ; also sheet 7,8,11,12
YEND7: 1F.17(3Q) ; also sheet 7,8,11,12
YEND8: 1F.16(4Q) ; also sheet 7,8,11,12
YEND9: 1F.15(5Q) ; also sheet 7,8,11,12
YEND10: 1F.14(6Q) ; also sheet 7,8,11,12
YEND11: 1F.13(7Q) ; also sheet 7,8,11,12
YEND12: 1F.12(8Q) ; also sheet 7,8,11,12
Unconnected: 1C.6(5D) 1C.7(6D) 1C.8(7D) 1C.9(8D) 1C.12(8Q) 1C.13(7Q) 1C.14(6Q) 1C.15(5Q) 1D.2(1D) 1D.3(2D) 1D.4(3D) 1D.5(4D) 1D.16(4Q) 1D.17(3Q) 1D.18(2Q) 1D.19(1Q) 3H.12(MX/MN) 3H.13(RCO) 4H.3 4H.6 4H.9 4H.16 4H.17

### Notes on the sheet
- Latches, for stablilzing inputs.
- 2nd X coord (destination)
- LSB Bank 1
- 2nd Y coord (destination) | Always Y2
- Increases vector RAM pointer
- First X, Then Y, Then Z
- Brightness
- Vector Counters: 2.5MHZ
- Vector Math Logic: 20MHZ

## Sheet 7 of 13: End Coordinate Latches
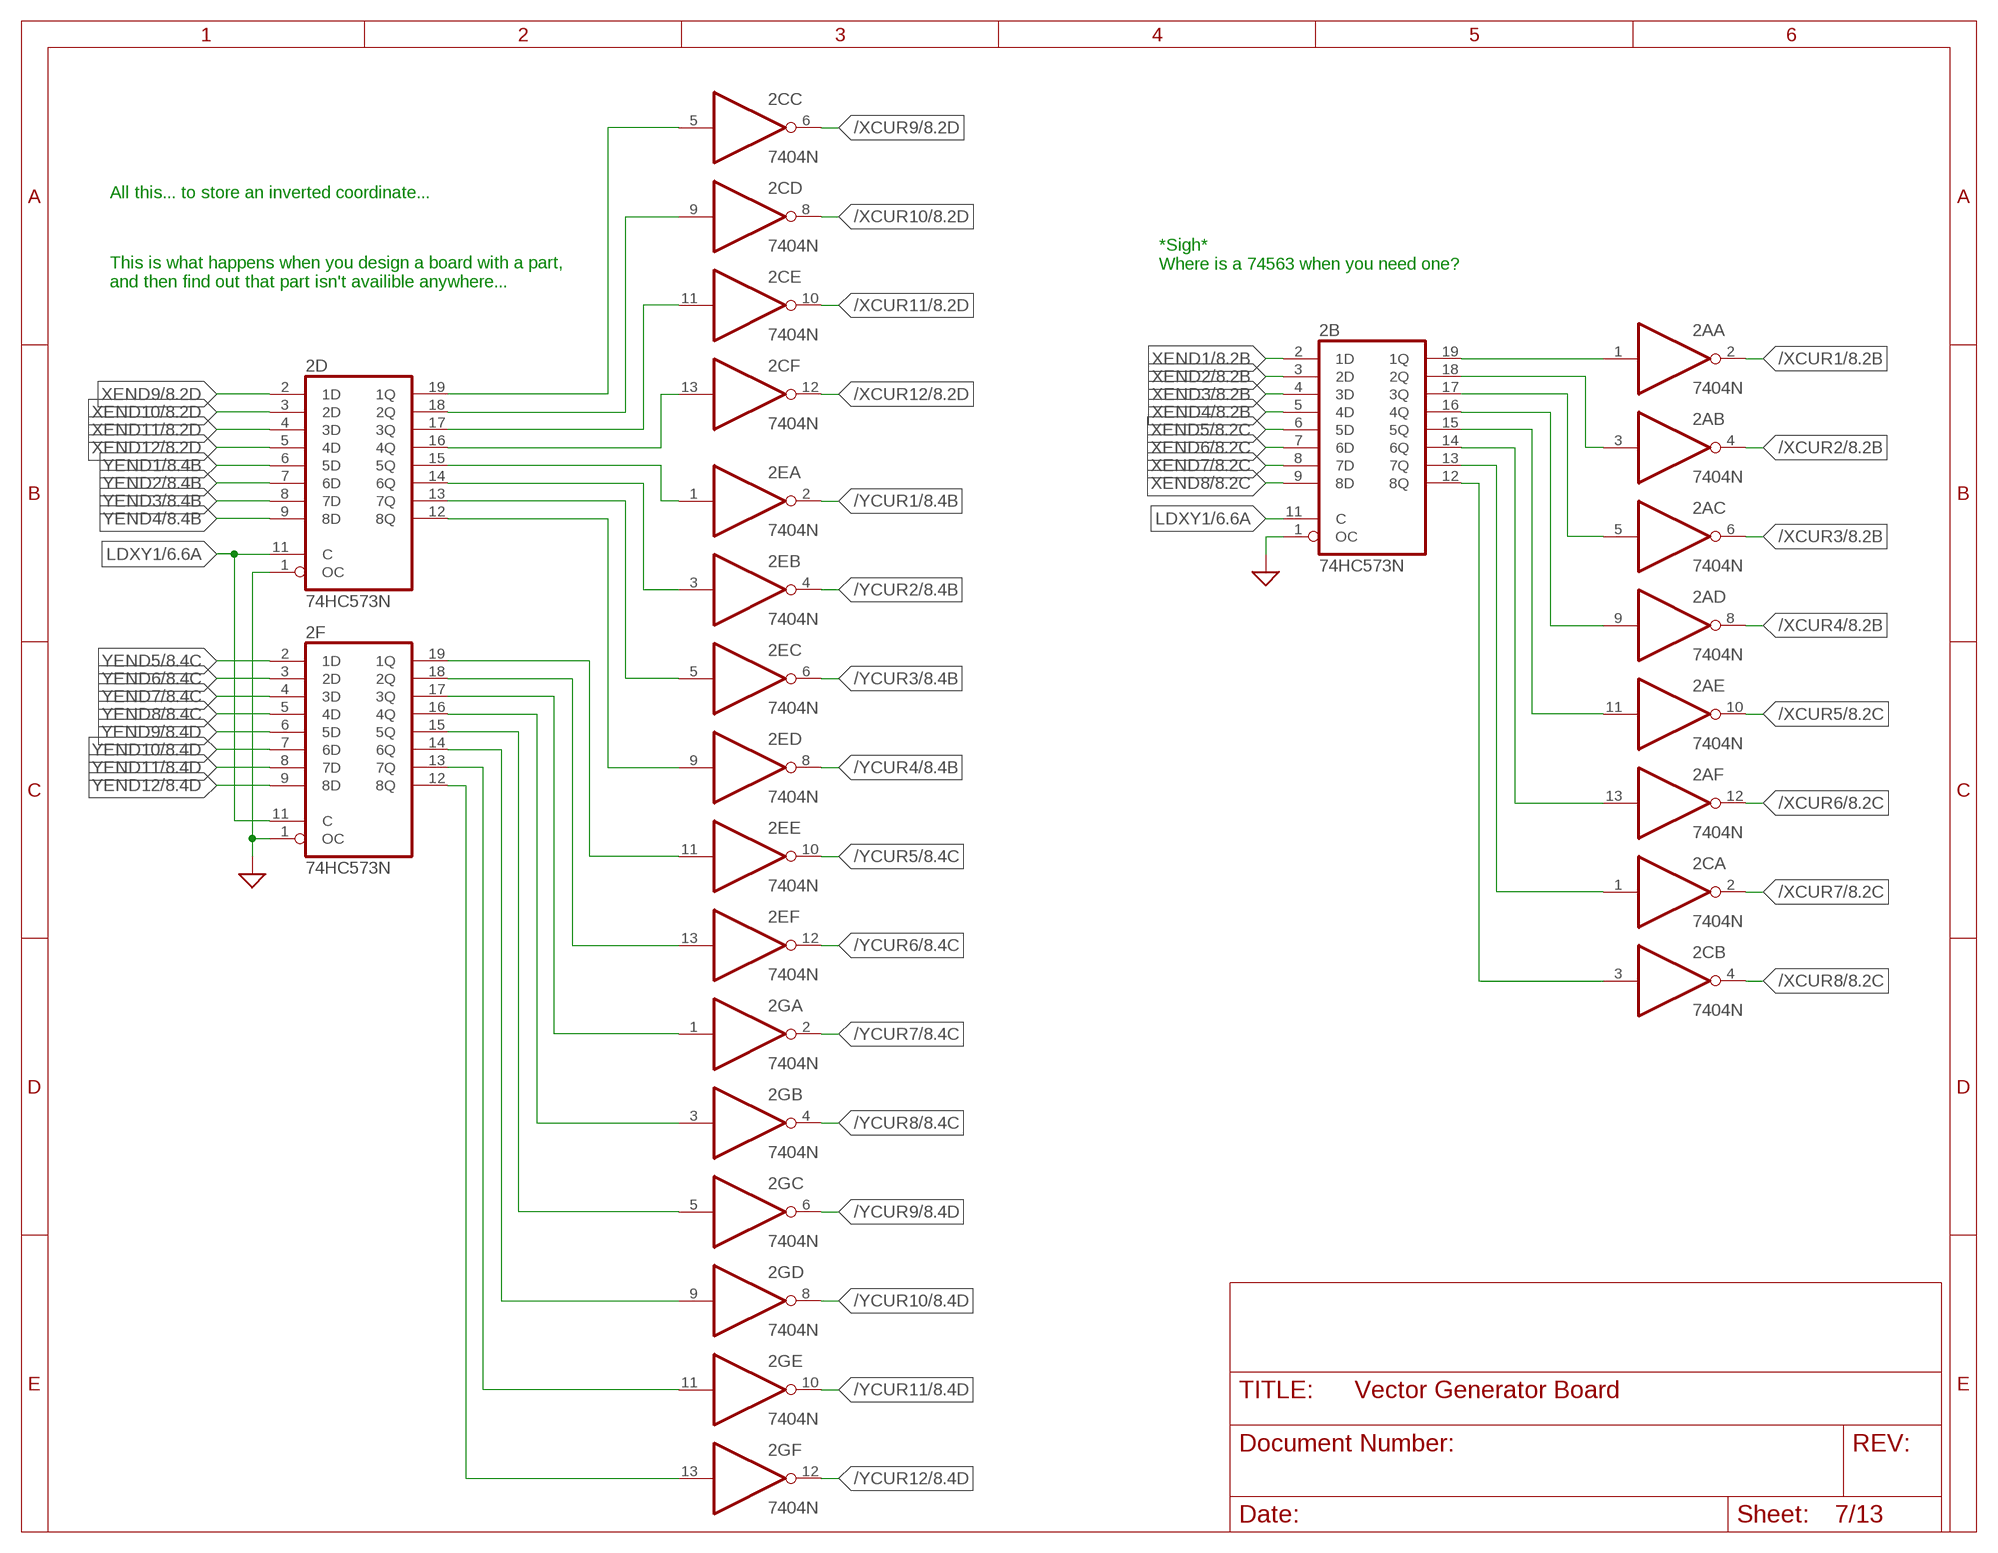
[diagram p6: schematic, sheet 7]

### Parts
2A  7404N  [DIL14]
2B  74HC573N  [DIL20]
2C  7404N  [DIL14]
2D  74HC573N  [DIL20]
2E  7404N  [DIL14]
2F  74HC573N  [DIL20]
2G  7404N  [DIL14]

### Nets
/XCUR1: 2A.2(A:O) ; also sheet 8
/XCUR2: 2A.4(B:O) ; also sheet 8
/XCUR3: 2A.6(C:O) ; also sheet 8
/XCUR4: 2A.8(D:O) ; also sheet 8
/XCUR5: 2A.10(E:O) ; also sheet 8
/XCUR6: 2A.12(F:O) ; also sheet 8
/XCUR7: 2C.2(A:O) ; also sheet 8
/XCUR8: 2C.4(B:O) ; also sheet 8
/XCUR9: 2C.6(C:O) ; also sheet 8
/XCUR10: 2C.8(D:O) ; also sheet 8
/XCUR11: 2C.10(E:O) ; also sheet 8
/XCUR12: 2C.12(F:O) ; also sheet 8
/YCUR1: 2E.2(A:O) ; also sheet 8
/YCUR2: 2E.4(B:O) ; also sheet 8
/YCUR3: 2E.6(C:O) ; also sheet 8
/YCUR4: 2E.8(D:O) ; also sheet 8
/YCUR5: 2E.10(E:O) ; also sheet 8
/YCUR6: 2E.12(F:O) ; also sheet 8
/YCUR7: 2G.2(A:O) ; also sheet 8
/YCUR8: 2G.4(B:O) ; also sheet 8
/YCUR9: 2G.6(C:O) ; also sheet 8
/YCUR10: 2G.8(D:O) ; also sheet 8
/YCUR11: 2G.10(E:O) ; also sheet 8
/YCUR12: 2G.12(F:O) ; also sheet 8
GND: 2B.1(OC) 2D.1(OC) 2F.1(OC) ; supply symbol labelled SUP ; also sheet 1,2,3,4,6,9,12,13
LDXY1: 2B.11(C) 2D.11(C) 2F.11(C) ; also sheet 6
N$58: 2A.1(A:I) 2B.19(1Q)
N$59: 2A.3(B:I) 2B.18(2Q)
N$60: 2A.5(C:I) 2B.17(3Q)
N$61: 2A.9(D:I) 2B.16(4Q)
N$62: 2A.11(E:I) 2B.15(5Q)
N$63: 2A.13(F:I) 2B.14(6Q)
N$64: 2B.13(7Q) 2C.1(A:I)
N$65: 2B.12(8Q) 2C.3(B:I)
N$66: 2C.5(C:I) 2D.19(1Q)
N$67: 2C.9(D:I) 2D.18(2Q)
N$68: 2C.11(E:I) 2D.17(3Q)
N$69: 2C.13(F:I) 2D.16(4Q)
N$70: 2D.15(5Q) 2E.1(A:I)
N$72: 2D.14(6Q) 2E.3(B:I)
N$73: 2D.13(7Q) 2E.5(C:I)
N$74: 2D.12(8Q) 2E.9(D:I)
N$75: 2F.12(8Q) 2G.13(F:I)
N$76: 2F.13(7Q) 2G.11(E:I)
N$77: 2F.14(6Q) 2G.9(D:I)
N$78: 2F.15(5Q) 2G.5(C:I)
N$93: 2F.16(4Q) 2G.3(B:I)
N$94: 2F.17(3Q) 2G.1(A:I)
N$95: 2E.13(F:I) 2F.18(2Q)
N$96: 2E.11(E:I) 2F.19(1Q)
XEND1: 2B.2(1D) ; also sheet 6,8,11,12
XEND2: 2B.3(2D) ; also sheet 6,8,11,12
XEND3: 2B.4(3D) ; also sheet 6,8,11,12
XEND4: 2B.5(4D) ; also sheet 6,8,11,12
XEND5: 2B.6(5D) ; also sheet 6,8,11,12
XEND6: 2B.7(6D) ; also sheet 6,8,11,12
XEND7: 2B.8(7D) ; also sheet 6,8,11,12
XEND8: 2B.9(8D) ; also sheet 6,8,11,12
XEND9: 2D.2(1D) ; also sheet 6,8,11,12
XEND10: 2D.3(2D) ; also sheet 6,8,11,12
XEND11: 2D.4(3D) ; also sheet 6,8,11,12
XEND12: 2D.5(4D) ; also sheet 6,8,11,12
YEND1: 2D.6(5D) ; also sheet 6,8,11,12
YEND2: 2D.7(6D) ; also sheet 6,8,11,12
YEND3: 2D.8(7D) ; also sheet 6,8,11,12
YEND4: 2D.9(8D) ; also sheet 6,8,11,12
YEND5: 2F.2(1D) ; also sheet 6,8,11,12
YEND6: 2F.3(2D) ; also sheet 6,8,11,12
YEND7: 2F.4(3D) ; also sheet 6,8,11,12
YEND8: 2F.5(4D) ; also sheet 6,8,11,12
YEND9: 2F.6(5D) ; also sheet 6,8,11,12
YEND10: 2F.7(6D) ; also sheet 6,8,11,12
YEND11: 2F.8(7D) ; also sheet 6,8,11,12
YEND12: 2F.9(8D) ; also sheet 6,8,11,12

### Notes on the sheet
- All this... to store an inverted coordinate...
- *Sigh*
  Where is a 74563 when you need one?
- This is what happens when you design a board with a part,
  and then find out that part isn't availible anywhere...

## Sheet 8 of 13: dY & dX Subtractor
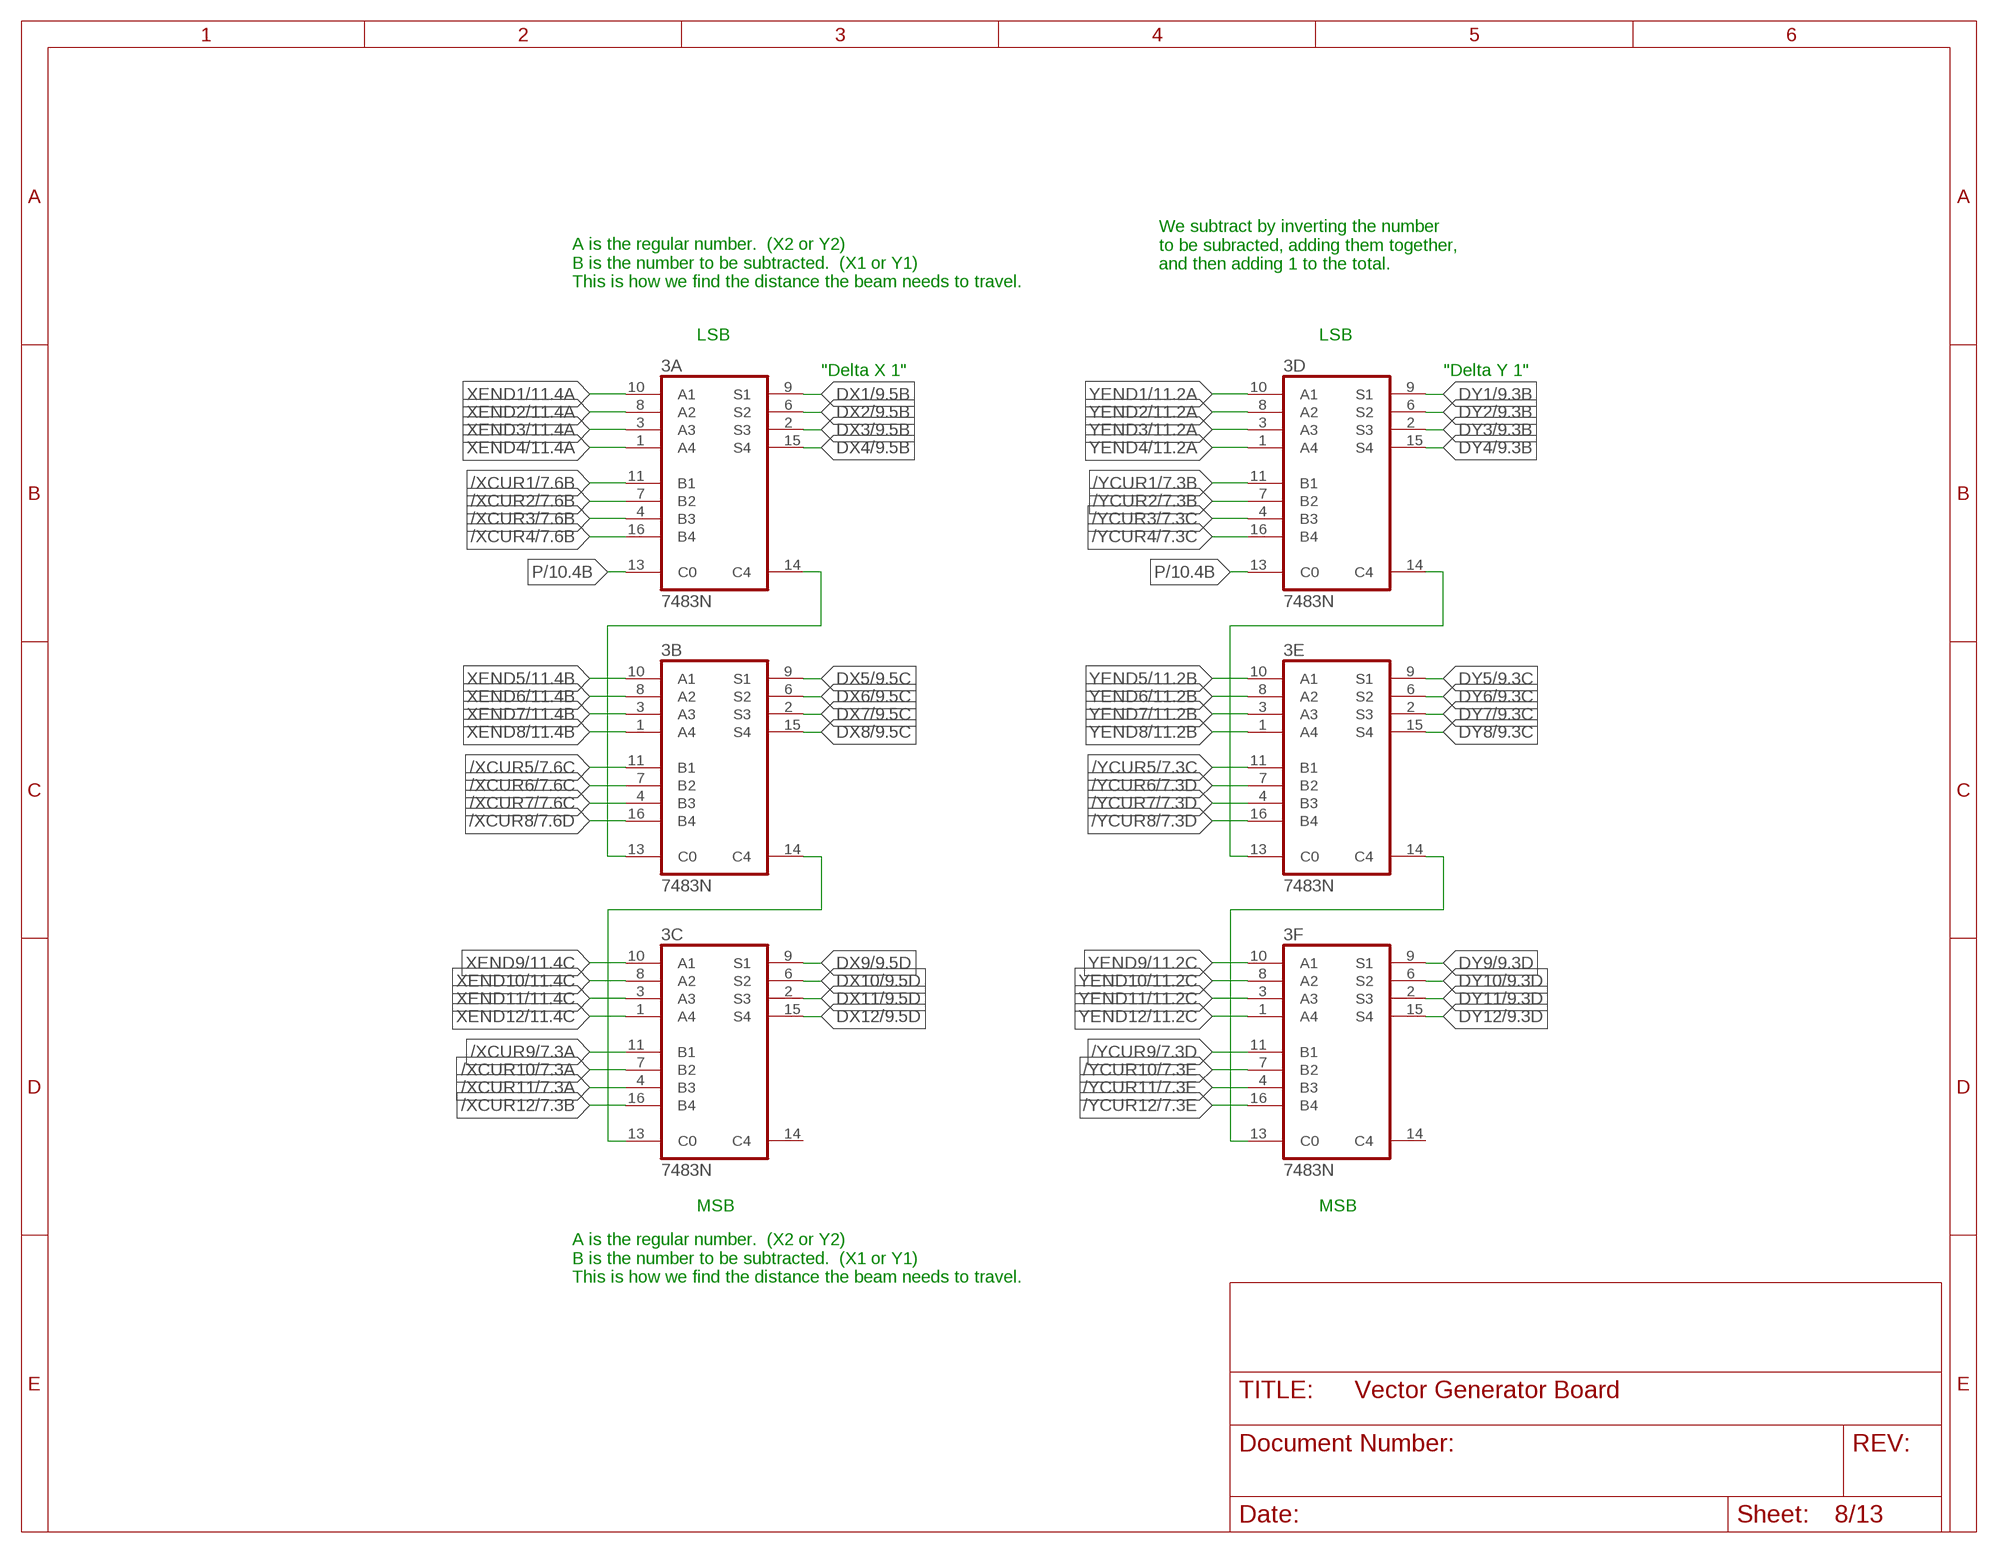
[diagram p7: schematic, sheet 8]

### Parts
3A  7483N  [DIL16]
3B  7483N  [DIL16]
3C  7483N  [DIL16]
3D  7483N  [DIL16]
3E  7483N  [DIL16]
3F  7483N  [DIL16]

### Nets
/XCUR1: 3A.11(B1) ; also sheet 7
/XCUR2: 3A.7(B2) ; also sheet 7
/XCUR3: 3A.4(B3) ; also sheet 7
/XCUR4: 3A.16(B4) ; also sheet 7
/XCUR5: 3B.11(B1) ; also sheet 7
/XCUR6: 3B.7(B2) ; also sheet 7
/XCUR7: 3B.4(B3) ; also sheet 7
/XCUR8: 3B.16(B4) ; also sheet 7
/XCUR9: 3C.11(B1) ; also sheet 7
/XCUR10: 3C.7(B2) ; also sheet 7
/XCUR11: 3C.4(B3) ; also sheet 7
/XCUR12: 3C.16(B4) ; also sheet 7
/YCUR1: 3D.11(B1) ; also sheet 7
/YCUR2: 3D.7(B2) ; also sheet 7
/YCUR3: 3D.4(B3) ; also sheet 7
/YCUR4: 3D.16(B4) ; also sheet 7
/YCUR5: 3E.11(B1) ; also sheet 7
/YCUR6: 3E.7(B2) ; also sheet 7
/YCUR7: 3E.4(B3) ; also sheet 7
/YCUR8: 3E.16(B4) ; also sheet 7
/YCUR9: 3F.11(B1) ; also sheet 7
/YCUR10: 3F.7(B2) ; also sheet 7
/YCUR11: 3F.4(B3) ; also sheet 7
/YCUR12: 3F.16(B4) ; also sheet 7
DX1: 3A.9(S1) ; also sheet 9
DX2: 3A.6(S2) ; also sheet 9
DX3: 3A.2(S3) ; also sheet 9
DX4: 3A.15(S4) ; also sheet 9
DX5: 3B.9(S1) ; also sheet 9
DX6: 3B.6(S2) ; also sheet 9
DX7: 3B.2(S3) ; also sheet 9
DX8: 3B.15(S4) ; also sheet 9
DX9: 3C.9(S1) ; also sheet 9
DX10: 3C.6(S2) ; also sheet 9
DX11: 3C.2(S3) ; also sheet 9
DX12: 3C.15(S4) ; also sheet 9
DY1: 3D.9(S1) ; also sheet 9
DY2: 3D.6(S2) ; also sheet 9
DY3: 3D.2(S3) ; also sheet 9
DY4: 3D.15(S4) ; also sheet 9
DY5: 3E.9(S1) ; also sheet 9
DY6: 3E.6(S2) ; also sheet 9
DY7: 3E.2(S3) ; also sheet 9
DY8: 3E.15(S4) ; also sheet 9
DY9: 3F.9(S1) ; also sheet 9
DY10: 3F.6(S2) ; also sheet 9
DY11: 3F.2(S3) ; also sheet 9
DY12: 3F.15(S4) ; also sheet 9
N$101: 3D.14(C4) 3E.13(C0)
N$102: 3E.14(C4) 3F.13(C0)
N$129: 3A.14(C4) 3B.13(C0)
N$155: 3B.14(C4) 3C.13(C0)
P: 3A.13(C0) 3D.13(C0) ; also sheet 1,10,11,12
XEND1: 3A.10(A1) ; also sheet 6,7,11,12
XEND2: 3A.8(A2) ; also sheet 6,7,11,12
XEND3: 3A.3(A3) ; also sheet 6,7,11,12
XEND4: 3A.1(A4) ; also sheet 6,7,11,12
XEND5: 3B.10(A1) ; also sheet 6,7,11,12
XEND6: 3B.8(A2) ; also sheet 6,7,11,12
XEND7: 3B.3(A3) ; also sheet 6,7,11,12
XEND8: 3B.1(A4) ; also sheet 6,7,11,12
XEND9: 3C.10(A1) ; also sheet 6,7,11,12
XEND10: 3C.8(A2) ; also sheet 6,7,11,12
XEND11: 3C.3(A3) ; also sheet 6,7,11,12
XEND12: 3C.1(A4) ; also sheet 6,7,11,12
YEND1: 3D.10(A1) ; also sheet 6,7,11,12
YEND2: 3D.8(A2) ; also sheet 6,7,11,12
YEND3: 3D.3(A3) ; also sheet 6,7,11,12
YEND4: 3D.1(A4) ; also sheet 6,7,11,12
YEND5: 3E.10(A1) ; also sheet 6,7,11,12
YEND6: 3E.8(A2) ; also sheet 6,7,11,12
YEND7: 3E.3(A3) ; also sheet 6,7,11,12
YEND8: 3E.1(A4) ; also sheet 6,7,11,12
YEND9: 3F.10(A1) ; also sheet 6,7,11,12
YEND10: 3F.8(A2) ; also sheet 6,7,11,12
YEND11: 3F.3(A3) ; also sheet 6,7,11,12
YEND12: 3F.1(A4) ; also sheet 6,7,11,12
Unconnected: 3C.14(C4) 3F.14(C4)

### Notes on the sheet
- We subtract by inverting the number 
  to be subracted, adding them together,
  and then adding 1 to the total.
- A is the regular number.  (X2 or Y2)
  B is the number to be subtracted.  (X1 or Y1)
  This is how we find the distance the beam needs to travel.
- LSB | LSB
- "Delta X 1" | "Delta Y 1"
- MSB | MSB
- A is the regular number.  (X2 or Y2)
  B is the number to be subtracted.  (X1 or Y1)
  This is how we find the distance the beam needs to travel.

## Sheet 9 of 13: Magnitude Incrementer
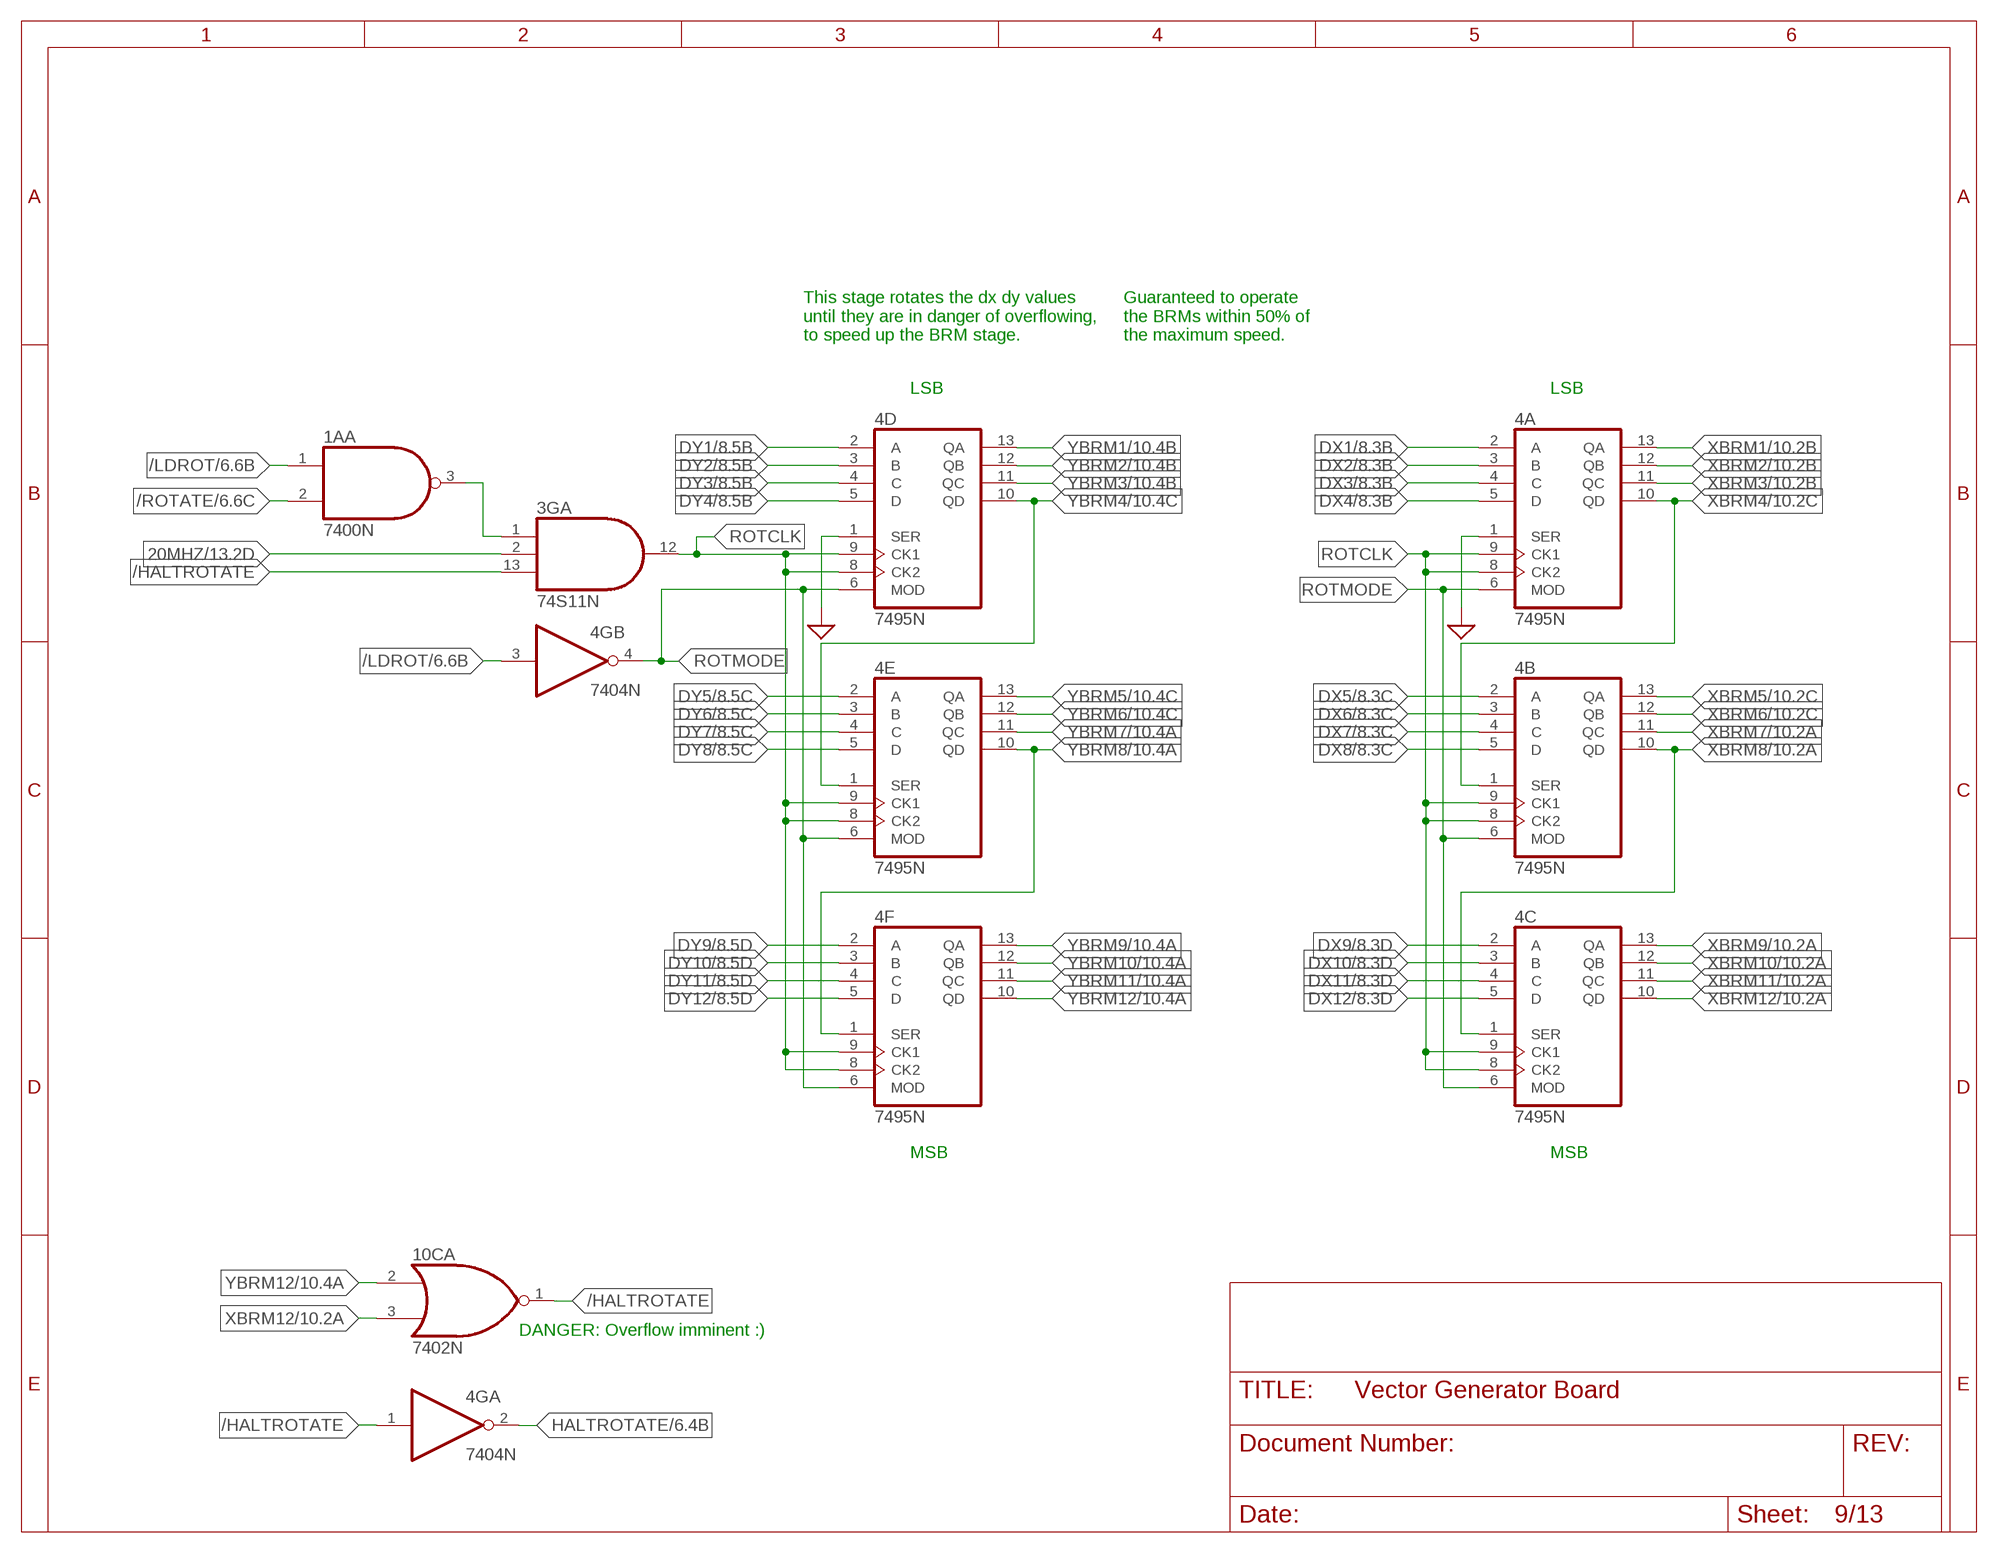
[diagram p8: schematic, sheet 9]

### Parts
1A  7400N  [DIL14]
4A  7495N  [DIL14]
4B  7495N  [DIL14]
4C  7495N  [DIL14]
4D  7495N  [DIL14]
4E  7495N  [DIL14]
4F  7495N  [DIL14]
10C  7402N  [DIL14]

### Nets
20MHZ: 3G.2(A:I1) ; also sheet 6,13
/HALTROTATE: 3G.13(A:I2) 4G.1(A:I) 10C.1(A:O)
/LDROT: 1A.1(A:I0) 4G.3(B:I) ; also sheet 6
/ROTATE: 1A.2(A:I1) ; also sheet 6
DX1: 4A.2(A) ; also sheet 8
DX2: 4A.3(B) ; also sheet 8
DX3: 4A.4(C) ; also sheet 8
DX4: 4A.5(D) ; also sheet 8
DX5: 4B.2(A) ; also sheet 8
DX6: 4B.3(B) ; also sheet 8
DX7: 4B.4(C) ; also sheet 8
DX8: 4B.5(D) ; also sheet 8
DX9: 4C.2(A) ; also sheet 8
DX10: 4C.3(B) ; also sheet 8
DX11: 4C.4(C) ; also sheet 8
DX12: 4C.5(D) ; also sheet 8
DY1: 4D.2(A) ; also sheet 8
DY2: 4D.3(B) ; also sheet 8
DY3: 4D.4(C) ; also sheet 8
DY4: 4D.5(D) ; also sheet 8
DY5: 4E.2(A) ; also sheet 8
DY6: 4E.3(B) ; also sheet 8
DY7: 4E.4(C) ; also sheet 8
DY8: 4E.5(D) ; also sheet 8
DY9: 4F.2(A) ; also sheet 8
DY10: 4F.3(B) ; also sheet 8
DY11: 4F.4(C) ; also sheet 8
DY12: 4F.5(D) ; also sheet 8
GND: 4A.1(SER) 4D.1(SER) ; supply symbol labelled SUP ; also sheet 1,2,3,4,6,7,12,13
HALTROTATE: 4G.2(A:O) ; also sheet 6
N$43: 1A.3(A:O) 3G.1(A:I0)
ROTCLK: 3G.12(A:O) 4A.8(CK2) 4A.9(CK1) 4B.8(CK2) 4B.9(CK1) 4C.8(CK2) 4C.9(CK1) 4D.8(CK2) 4D.9(CK1) 4E.8(CK2) 4E.9(CK1) 4F.8(CK2) 4F.9(CK1)
ROTMODE: 4A.6(MOD) 4B.6(MOD) 4C.6(MOD) 4D.6(MOD) 4E.6(MOD) 4F.6(MOD) 4G.4(B:O)
XBRM1: 4A.13(QA) ; also sheet 10
XBRM2: 4A.12(QB) ; also sheet 10
XBRM3: 4A.11(QC) ; also sheet 10
XBRM4: 4A.10(QD) 4B.1(SER) ; also sheet 10
XBRM5: 4B.13(QA) ; also sheet 10
XBRM6: 4B.12(QB) ; also sheet 10
XBRM7: 4B.11(QC) ; also sheet 10
XBRM8: 4B.10(QD) 4C.1(SER) ; also sheet 10
XBRM9: 4C.13(QA) ; also sheet 10
XBRM10: 4C.12(QB) ; also sheet 10
XBRM11: 4C.11(QC) ; also sheet 10
XBRM12: 4C.10(QD) 10C.3(A:I1) ; also sheet 10
YBRM1: 4D.13(QA) ; also sheet 10
YBRM2: 4D.12(QB) ; also sheet 10
YBRM3: 4D.11(QC) ; also sheet 10
YBRM4: 4D.10(QD) 4E.1(SER) ; also sheet 10
YBRM5: 4E.13(QA) ; also sheet 10
YBRM6: 4E.12(QB) ; also sheet 10
YBRM7: 4E.11(QC) ; also sheet 10
YBRM8: 4E.10(QD) 4F.1(SER) ; also sheet 10
YBRM9: 4F.13(QA) ; also sheet 10
YBRM10: 4F.12(QB) ; also sheet 10
YBRM11: 4F.11(QC) ; also sheet 10
YBRM12: 4F.10(QD) 10C.2(A:I0) ; also sheet 10

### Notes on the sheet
- This stage rotates the dx dy values
  until they are in danger of overflowing,
  to speed up the BRM stage.
- Guaranteed to operate
  the BRMs within 50% of
  the maximum speed.
- LSB | LSB
- MSB | MSB
- DANGER: Overflow imminent :)

## Sheet 10 of 13: Binary Rate Multipliers
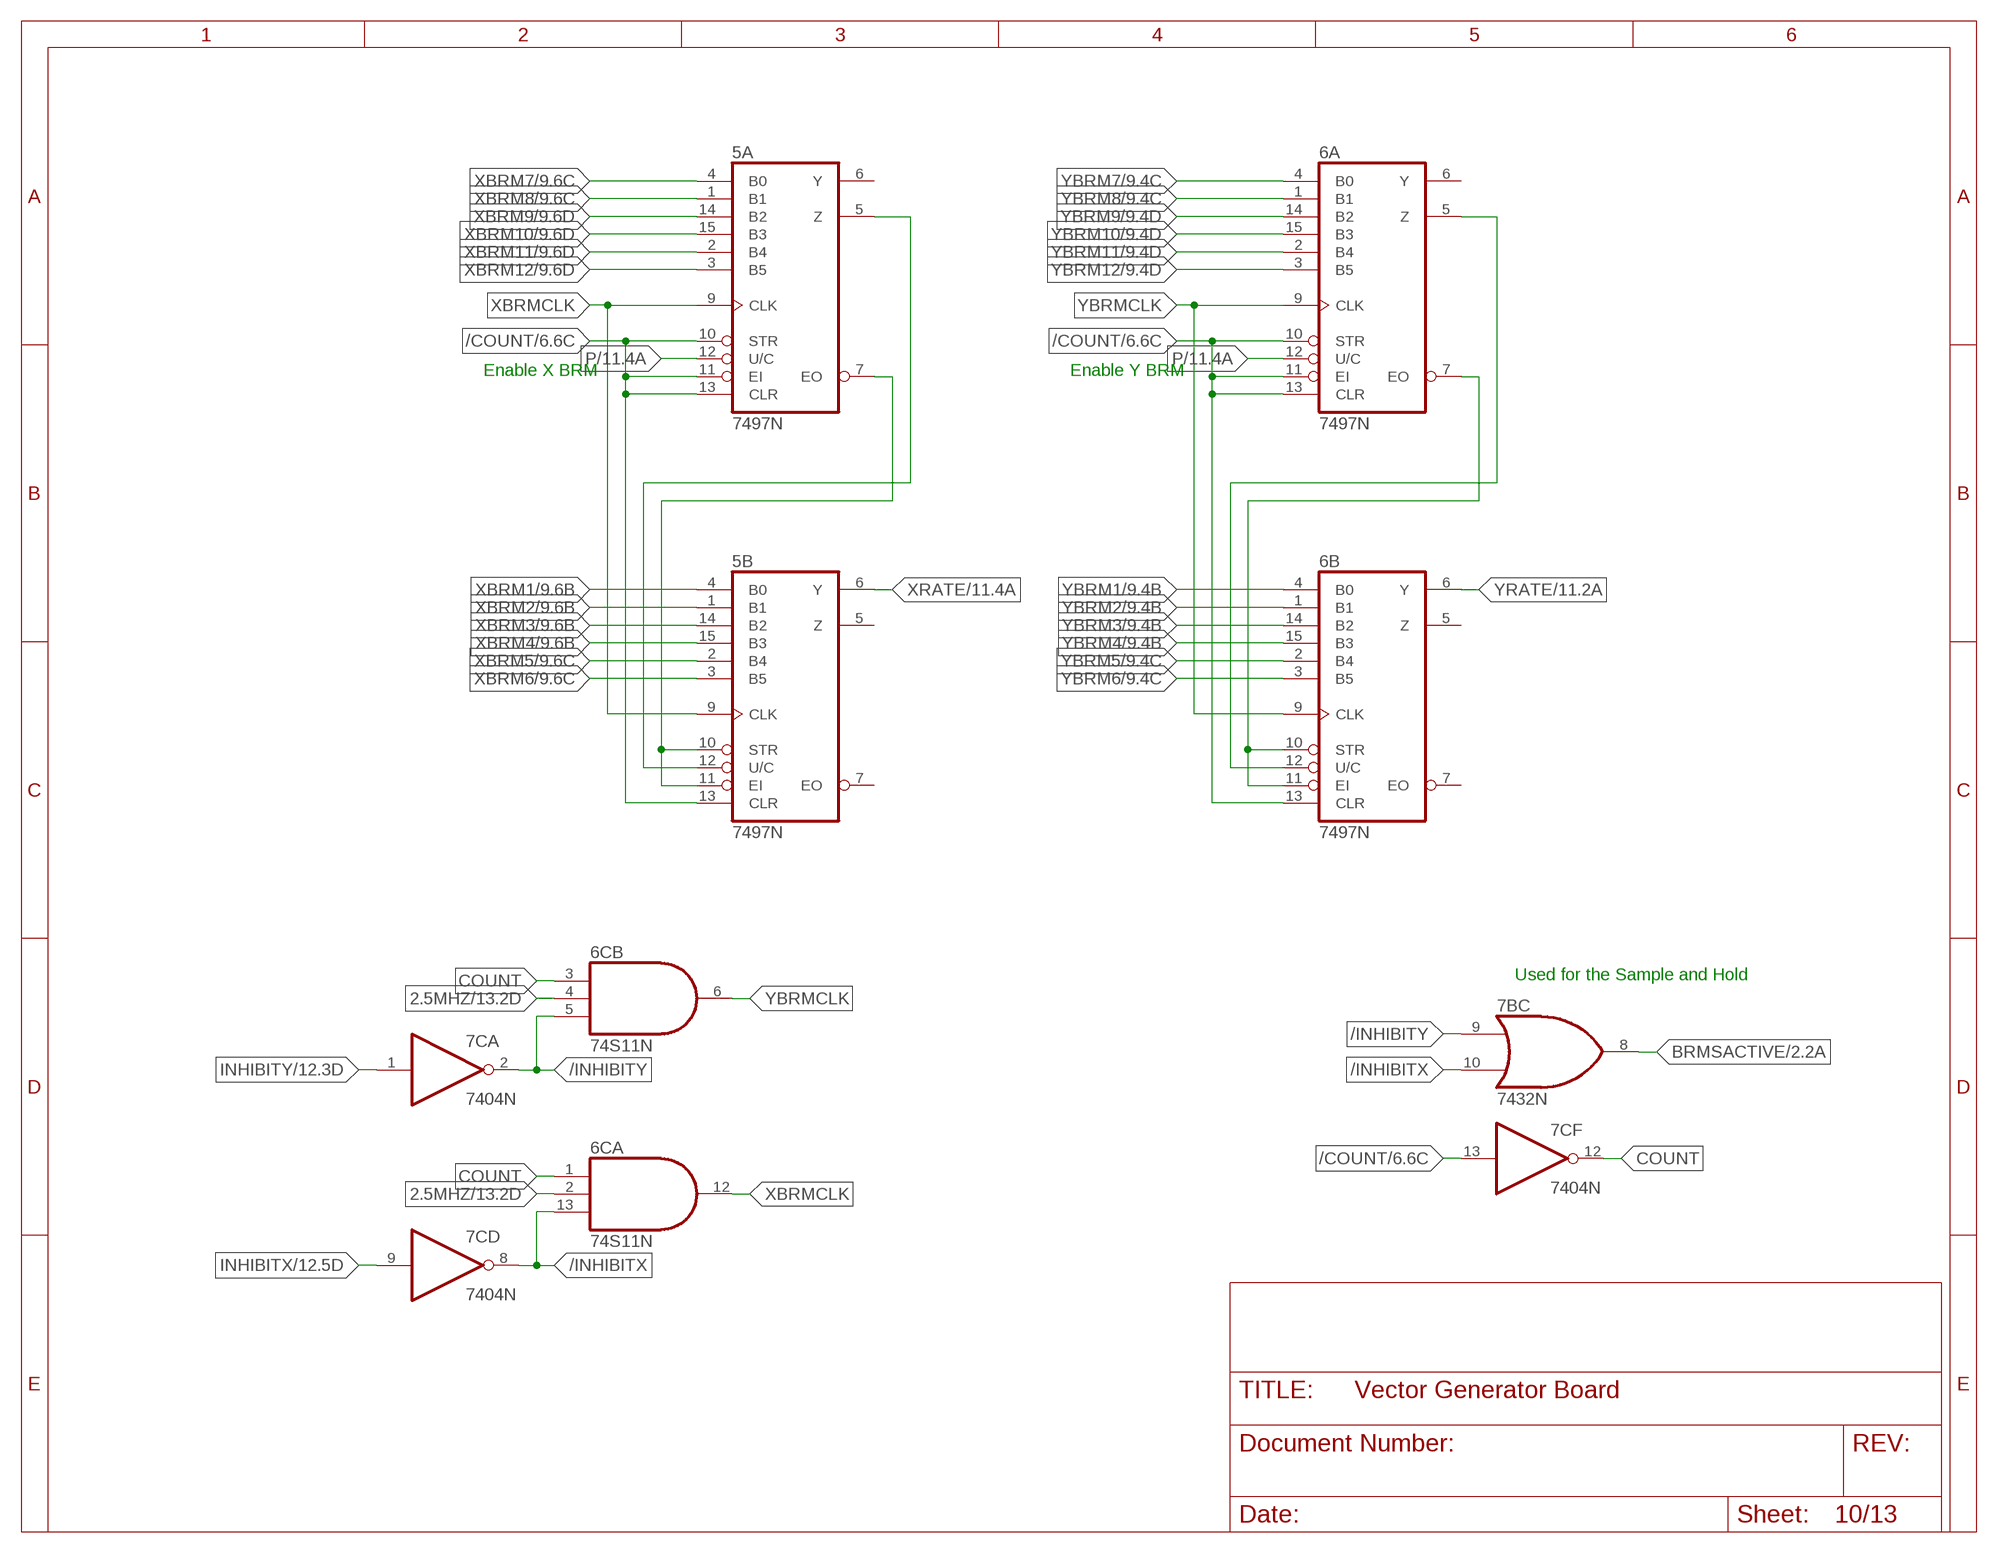
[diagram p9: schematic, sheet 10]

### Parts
5A  7497N  [DIL16]
5B  7497N  [DIL16]
6A  7497N  [DIL16]
6B  7497N  [DIL16]
6C  74S11N  [DIL14]
7B  7432N  [DIL14]
7C  7404N  [DIL14]

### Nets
2.5MHZ: 6C.2(A:I1) 6C.4(B:I1) ; also sheet 2,13
/COUNT: 5A.10(STR) 5A.11(EI) 5A.13(CLR) 5B.13(CLR) 6A.10(STR) 6A.11(EI) 6A.13(CLR) 6B.13(CLR) 7C.13(F:I) ; also sheet 6
/INHIBITX: 6C.13(A:I2) 7B.10(C:I1) 7C.8(D:O)
/INHIBITY: 6C.5(B:I2) 7B.9(C:I0) 7C.2(A:O)
BRMSACTIVE: 7B.8(C:O) ; also sheet 2
COUNT: 6C.1(A:I0) 6C.3(B:I0) 7C.12(F:O)
INHIBITX: 7C.9(D:I) ; also sheet 12
INHIBITY: 7C.1(A:I) ; also sheet 12
N$36: 5A.7(EO) 5B.10(STR) 5B.11(EI)
N$40: 5A.5(Z) 5B.12(U/C)
N$168: 6A.7(EO) 6B.10(STR) 6B.11(EI)
N$169: 6A.5(Z) 6B.12(U/C)
P: 5A.12(U/C) 6A.12(U/C) ; also sheet 1,8,11,12
XBRM1: 5B.4(B0) ; also sheet 9
XBRM2: 5B.1(B1) ; also sheet 9
XBRM3: 5B.14(B2) ; also sheet 9
XBRM4: 5B.15(B3) ; also sheet 9
XBRM5: 5B.2(B4) ; also sheet 9
XBRM6: 5B.3(B5) ; also sheet 9
XBRM7: 5A.4(B0) ; also sheet 9
XBRM8: 5A.1(B1) ; also sheet 9
XBRM9: 5A.14(B2) ; also sheet 9
XBRM10: 5A.15(B3) ; also sheet 9
XBRM11: 5A.2(B4) ; also sheet 9
XBRM12: 5A.3(B5) ; also sheet 9
XBRMCLK: 5A.9(CLK) 5B.9(CLK) 6C.12(A:O)
XRATE: 5B.6(Y) ; also sheet 11
YBRM1: 6B.4(B0) ; also sheet 9
YBRM2: 6B.1(B1) ; also sheet 9
YBRM3: 6B.14(B2) ; also sheet 9
YBRM4: 6B.15(B3) ; also sheet 9
YBRM5: 6B.2(B4) ; also sheet 9
YBRM6: 6B.3(B5) ; also sheet 9
YBRM7: 6A.4(B0) ; also sheet 9
YBRM8: 6A.1(B1) ; also sheet 9
YBRM9: 6A.14(B2) ; also sheet 9
YBRM10: 6A.15(B3) ; also sheet 9
YBRM11: 6A.2(B4) ; also sheet 9
YBRM12: 6A.3(B5) ; also sheet 9
YBRMCLK: 6A.9(CLK) 6B.9(CLK) 6C.6(B:O)
YRATE: 6B.6(Y) ; also sheet 11
Unconnected: 5A.6(Y) 5B.5(Z) 5B.7(EO) 6A.6(Y) 6B.5(Z) 6B.7(EO)

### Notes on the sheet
- Enable X BRM | Enable Y BRM
- Used for the Sample and Hold

## Sheet 11 of 13: X and Y Position Counters
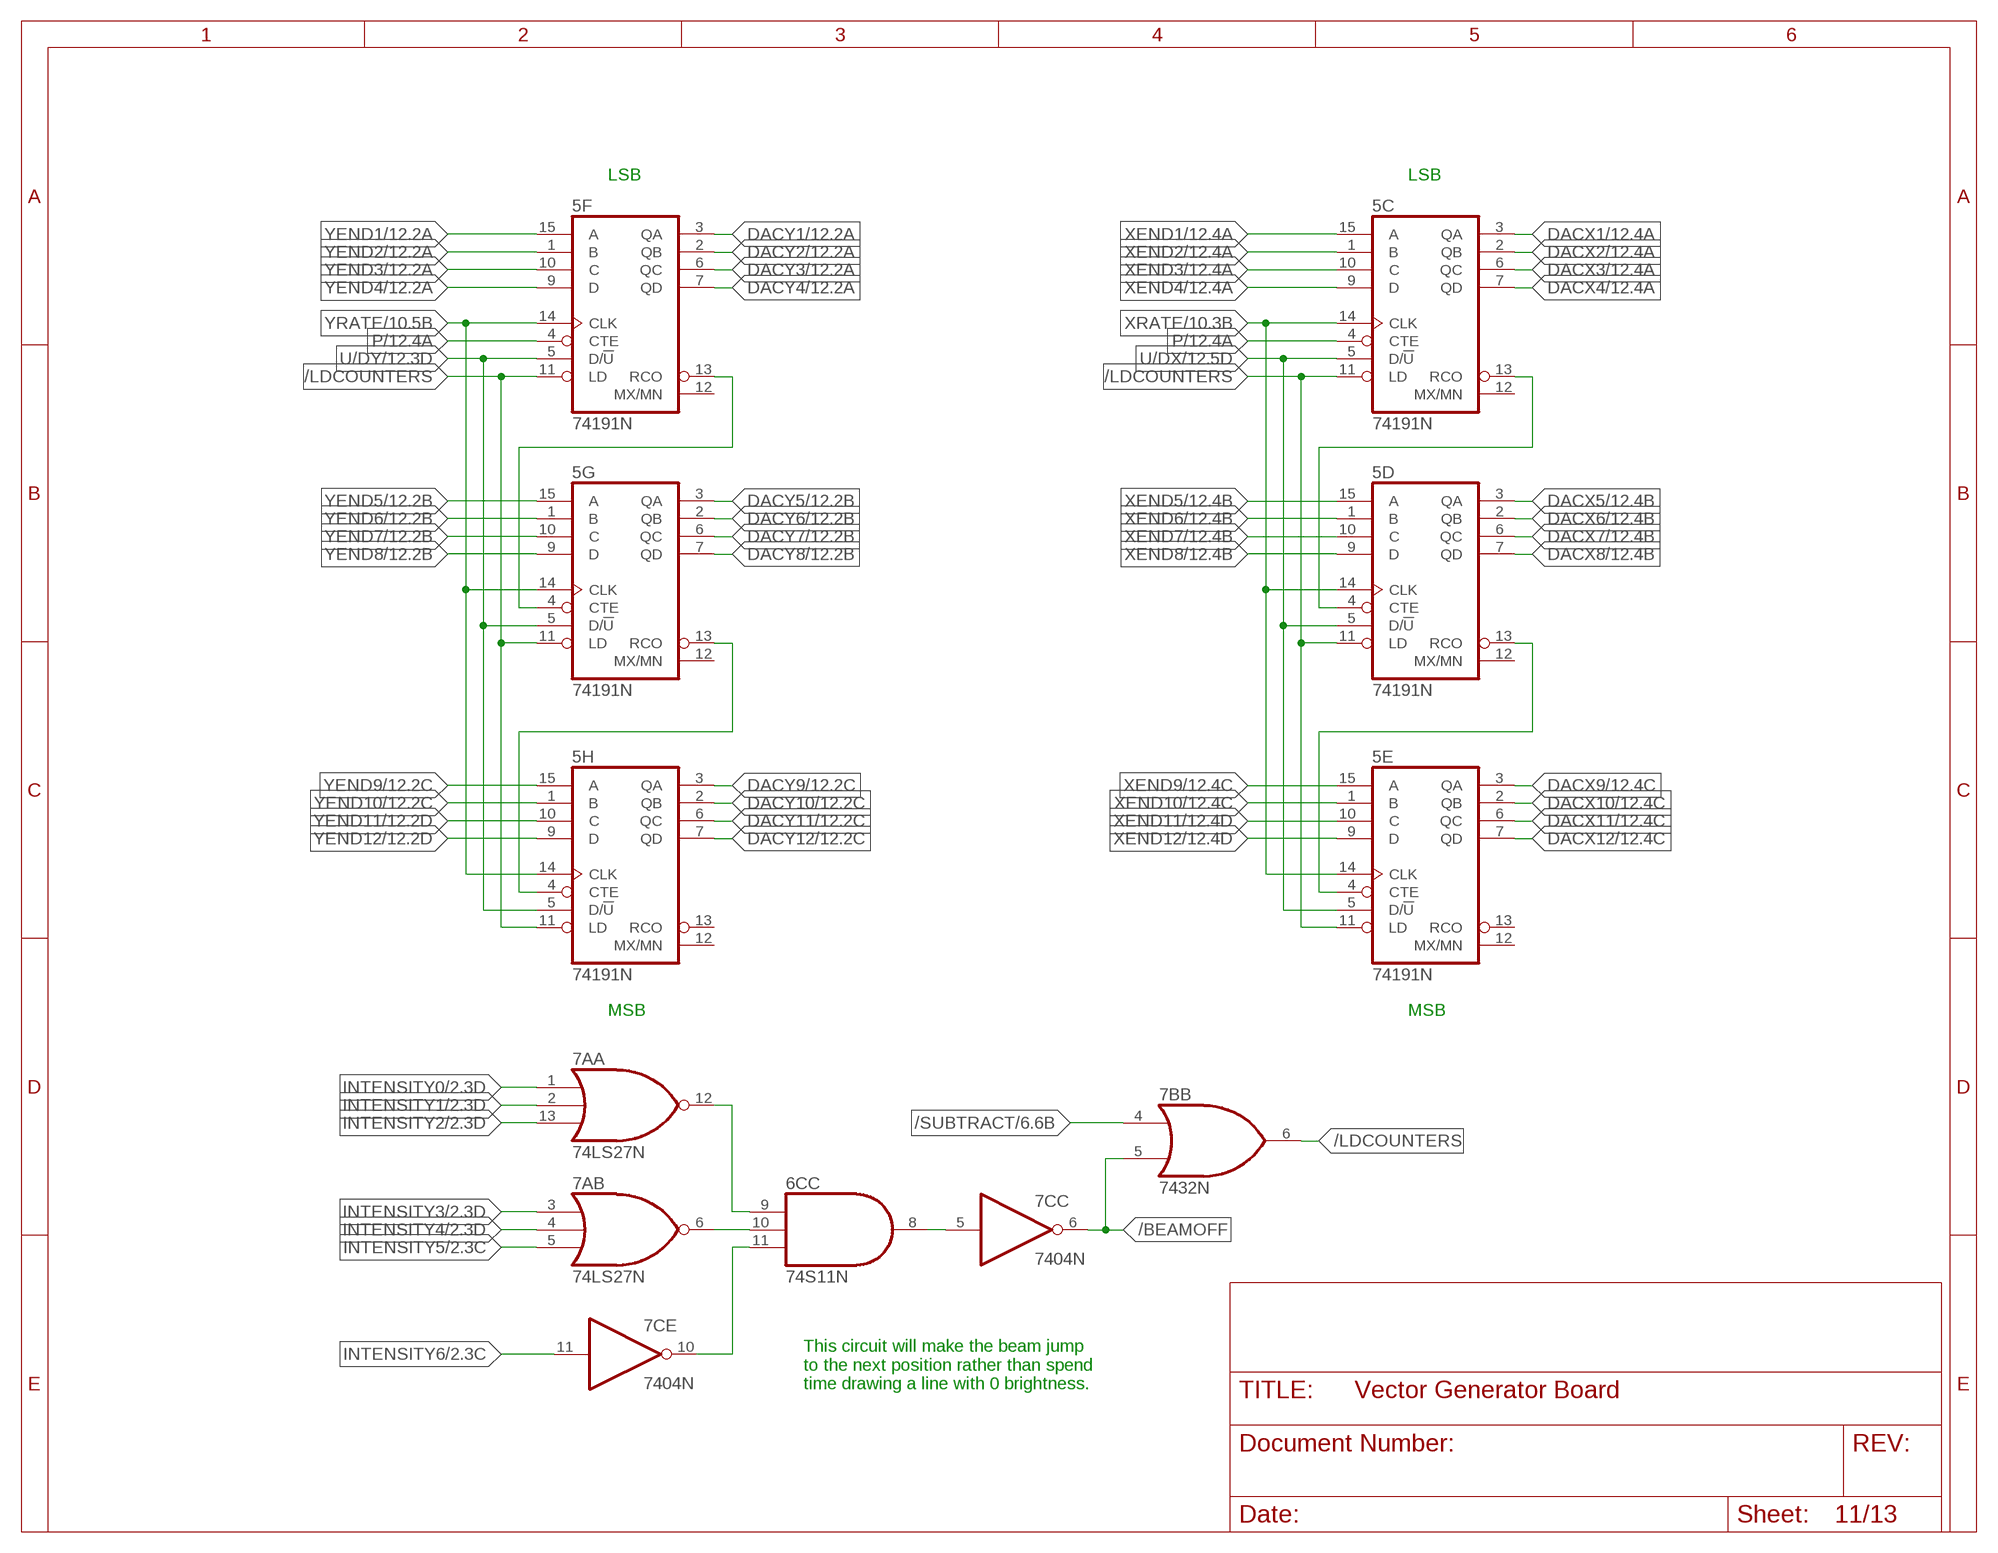
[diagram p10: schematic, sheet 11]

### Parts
5C  74191N  [DIL16]
5D  74191N  [DIL16]
5E  74191N  [DIL16]
5F  74191N  [DIL16]
5G  74191N  [DIL16]
5H  74191N  [DIL16]
7A  74LS27N  [DIL14]

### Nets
/BEAMOFF: 7B.5(B:I1) 7C.6(C:O)
/LDCOUNTERS: 5C.11(LD) 5D.11(LD) 5E.11(LD) 5F.11(LD) 5G.11(LD) 5H.11(LD) 7B.6(B:O)
/SUBTRACT: 7B.4(B:I0) ; also sheet 6
DACX1: 5C.3(QA) ; also sheet 3,12
DACX2: 5C.2(QB) ; also sheet 3,12
DACX3: 5C.6(QC) ; also sheet 3,12
DACX4: 5C.7(QD) ; also sheet 3,12
DACX5: 5D.3(QA) ; also sheet 3,12
DACX6: 5D.2(QB) ; also sheet 3,12
DACX7: 5D.6(QC) ; also sheet 3,12
DACX8: 5D.7(QD) ; also sheet 3,12
DACX9: 5E.3(QA) ; also sheet 3,12
DACX10: 5E.2(QB) ; also sheet 3,12
DACX11: 5E.6(QC) ; also sheet 3,12
DACX12: 5E.7(QD) ; also sheet 3,12
DACY1: 5F.3(QA) ; also sheet 4,12
DACY2: 5F.2(QB) ; also sheet 4,12
DACY3: 5F.6(QC) ; also sheet 4,12
DACY4: 5F.7(QD) ; also sheet 4,12
DACY5: 5G.3(QA) ; also sheet 4,12
DACY6: 5G.2(QB) ; also sheet 4,12
DACY7: 5G.6(QC) ; also sheet 4,12
DACY8: 5G.7(QD) ; also sheet 4,12
DACY9: 5H.3(QA) ; also sheet 4,12
DACY10: 5H.2(QB) ; also sheet 4,12
DACY11: 5H.6(QC) ; also sheet 4,12
DACY12: 5H.7(QD) ; also sheet 4,12
INTENSITY0: 7A.1(A:I0) ; also sheet 2,6
INTENSITY1: 7A.2(A:I1) ; also sheet 2,6
INTENSITY2: 7A.13(A:I2) ; also sheet 2,6
INTENSITY3: 7A.3(B:I0) ; also sheet 2,6
INTENSITY4: 7A.4(B:I1) ; also sheet 2,6
INTENSITY5: 7A.5(B:I2) ; also sheet 2,6
INTENSITY6: 7C.11(E:I) ; also sheet 2,6
N$41: 5C.13(RCO) 5D.4(CTE)
N$42: 5D.13(RCO) 5E.4(CTE)
N$79: 5F.13(RCO) 5G.4(CTE)
N$80: 5G.13(RCO) 5H.4(CTE)
N$138: 6C.8(C:O) 7C.5(C:I)
N$139: 6C.10(C:I1) 7A.6(B:O)
N$140: 6C.9(C:I0) 7A.12(A:O)
N$141: 6C.11(C:I2) 7C.10(E:O)
P: 5C.4(CTE) 5F.4(CTE) ; also sheet 1,8,10,12
U/DX: 5C.5(D/!U) 5D.5(D/!U) 5E.5(D/!U) ; also sheet 12
U/DY: 5F.5(D/!U) 5G.5(D/!U) 5H.5(D/!U) ; also sheet 12
XEND1: 5C.15(A) ; also sheet 6,7,8,12
XEND2: 5C.1(B) ; also sheet 6,7,8,12
XEND3: 5C.10(C) ; also sheet 6,7,8,12
XEND4: 5C.9(D) ; also sheet 6,7,8,12
XEND5: 5D.15(A) ; also sheet 6,7,8,12
XEND6: 5D.1(B) ; also sheet 6,7,8,12
XEND7: 5D.10(C) ; also sheet 6,7,8,12
XEND8: 5D.9(D) ; also sheet 6,7,8,12
XEND9: 5E.15(A) ; also sheet 6,7,8,12
XEND10: 5E.1(B) ; also sheet 6,7,8,12
XEND11: 5E.10(C) ; also sheet 6,7,8,12
XEND12: 5E.9(D) ; also sheet 6,7,8,12
XRATE: 5C.14(CLK) 5D.14(CLK) 5E.14(CLK) ; also sheet 10
YEND1: 5F.15(A) ; also sheet 6,7,8,12
YEND2: 5F.1(B) ; also sheet 6,7,8,12
YEND3: 5F.10(C) ; also sheet 6,7,8,12
YEND4: 5F.9(D) ; also sheet 6,7,8,12
YEND5: 5G.15(A) ; also sheet 6,7,8,12
YEND6: 5G.1(B) ; also sheet 6,7,8,12
YEND7: 5G.10(C) ; also sheet 6,7,8,12
YEND8: 5G.9(D) ; also sheet 6,7,8,12
YEND9: 5H.15(A) ; also sheet 6,7,8,12
YEND10: 5H.1(B) ; also sheet 6,7,8,12
YEND11: 5H.10(C) ; also sheet 6,7,8,12
YEND12: 5H.9(D) ; also sheet 6,7,8,12
YRATE: 5F.14(CLK) 5G.14(CLK) 5H.14(CLK) ; also sheet 10
Unconnected: 5C.12(MX/MN) 5D.12(MX/MN) 5E.12(MX/MN) 5E.13(RCO) 5F.12(MX/MN) 5G.12(MX/MN) 5H.12(MX/MN) 5H.13(RCO)

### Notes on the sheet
- LSB | LSB
- MSB | MSB
- This circuit will make the beam jump
  to the next position rather than spend
  time drawing a line with 0 brightness.

## Sheet 12 of 13: X and Y Position Comparators
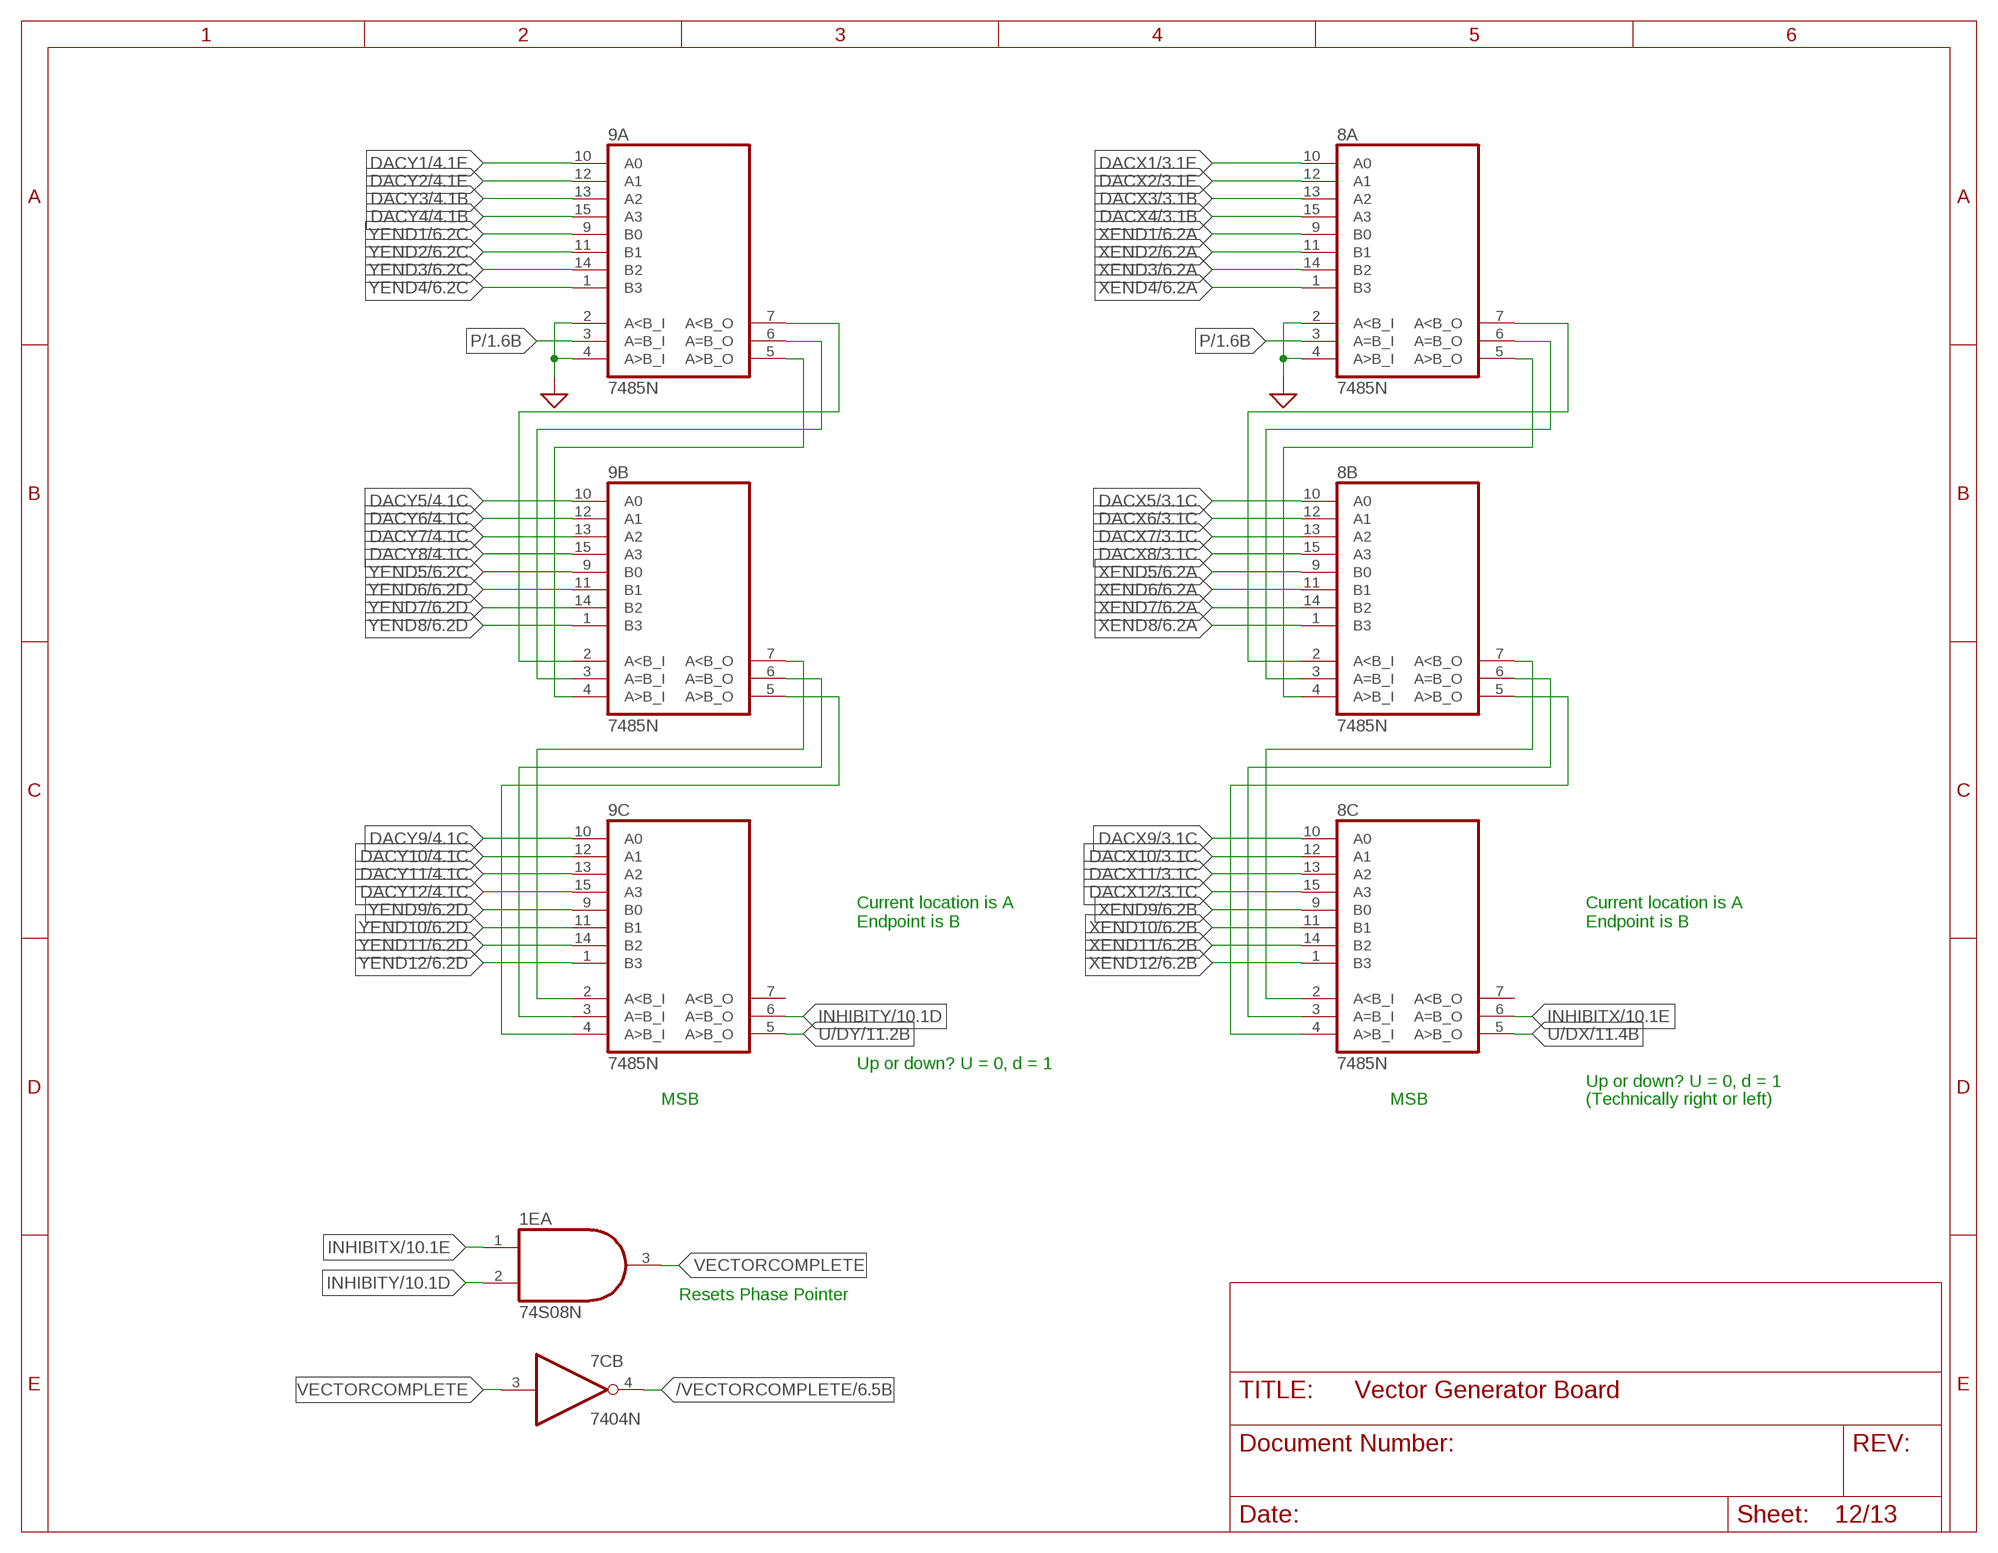
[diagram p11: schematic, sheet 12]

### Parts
8A  7485N  [DIL16]
8B  7485N  [DIL16]
8C  7485N  [DIL16]
9A  7485N  [DIL16]
9B  7485N  [DIL16]
9C  7485N  [DIL16]

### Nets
/VECTORCOMPLETE: 7C.4(B:O) ; also sheet 6
DACX1: 8A.10(A0) ; also sheet 3,11
DACX2: 8A.12(A1) ; also sheet 3,11
DACX3: 8A.13(A2) ; also sheet 3,11
DACX4: 8A.15(A3) ; also sheet 3,11
DACX5: 8B.10(A0) ; also sheet 3,11
DACX6: 8B.12(A1) ; also sheet 3,11
DACX7: 8B.13(A2) ; also sheet 3,11
DACX8: 8B.15(A3) ; also sheet 3,11
DACX9: 8C.10(A0) ; also sheet 3,11
DACX10: 8C.12(A1) ; also sheet 3,11
DACX11: 8C.13(A2) ; also sheet 3,11
DACX12: 8C.15(A3) ; also sheet 3,11
DACY1: 9A.10(A0) ; also sheet 4,11
DACY2: 9A.12(A1) ; also sheet 4,11
DACY3: 9A.13(A2) ; also sheet 4,11
DACY4: 9A.15(A3) ; also sheet 4,11
DACY5: 9B.10(A0) ; also sheet 4,11
DACY6: 9B.12(A1) ; also sheet 4,11
DACY7: 9B.13(A2) ; also sheet 4,11
DACY8: 9B.15(A3) ; also sheet 4,11
DACY9: 9C.10(A0) ; also sheet 4,11
DACY10: 9C.12(A1) ; also sheet 4,11
DACY11: 9C.13(A2) ; also sheet 4,11
DACY12: 9C.15(A3) ; also sheet 4,11
GND: 8A.2(A<B_I) 8A.4(A>B_I) 9A.2(A<B_I) 9A.4(A>B_I) ; supply symbol labelled SUP ; also sheet 1,2,3,4,6,7,9,13
INHIBITX: 1E.1(A:I0) 8C.6(A=B_O) ; also sheet 10
INHIBITY: 1E.2(A:I1) 9C.6(A=B_O) ; also sheet 10
N$81: 9B.7(A<B_O) 9C.2(A<B_I)
N$82: 9B.6(A=B_O) 9C.3(A=B_I)
N$83: 9B.5(A>B_O) 9C.4(A>B_I)
N$84: 9A.7(A<B_O) 9B.2(A<B_I)
N$85: 9A.6(A=B_O) 9B.3(A=B_I)
N$86: 9A.5(A>B_O) 9B.4(A>B_I)
N$87: 8B.7(A<B_O) 8C.2(A<B_I)
N$88: 8B.6(A=B_O) 8C.3(A=B_I)
N$89: 8B.5(A>B_O) 8C.4(A>B_I)
N$90: 8A.7(A<B_O) 8B.2(A<B_I)
N$91: 8A.6(A=B_O) 8B.3(A=B_I)
N$92: 8A.5(A>B_O) 8B.4(A>B_I)
P: 8A.3(A=B_I) 9A.3(A=B_I) ; also sheet 1,8,10,11
U/DX: 8C.5(A>B_O) ; also sheet 11
U/DY: 9C.5(A>B_O) ; also sheet 11
VECTORCOMPLETE: 1E.3(A:O) 7C.3(B:I)
XEND1: 8A.9(B0) ; also sheet 6,7,8,11
XEND2: 8A.11(B1) ; also sheet 6,7,8,11
XEND3: 8A.14(B2) ; also sheet 6,7,8,11
XEND4: 8A.1(B3) ; also sheet 6,7,8,11
XEND5: 8B.9(B0) ; also sheet 6,7,8,11
XEND6: 8B.11(B1) ; also sheet 6,7,8,11
XEND7: 8B.14(B2) ; also sheet 6,7,8,11
XEND8: 8B.1(B3) ; also sheet 6,7,8,11
XEND9: 8C.9(B0) ; also sheet 6,7,8,11
XEND10: 8C.11(B1) ; also sheet 6,7,8,11
XEND11: 8C.14(B2) ; also sheet 6,7,8,11
XEND12: 8C.1(B3) ; also sheet 6,7,8,11
YEND1: 9A.9(B0) ; also sheet 6,7,8,11
YEND2: 9A.11(B1) ; also sheet 6,7,8,11
YEND3: 9A.14(B2) ; also sheet 6,7,8,11
YEND4: 9A.1(B3) ; also sheet 6,7,8,11
YEND5: 9B.9(B0) ; also sheet 6,7,8,11
YEND6: 9B.11(B1) ; also sheet 6,7,8,11
YEND7: 9B.14(B2) ; also sheet 6,7,8,11
YEND8: 9B.1(B3) ; also sheet 6,7,8,11
YEND9: 9C.9(B0) ; also sheet 6,7,8,11
YEND10: 9C.11(B1) ; also sheet 6,7,8,11
YEND11: 9C.14(B2) ; also sheet 6,7,8,11
YEND12: 9C.1(B3) ; also sheet 6,7,8,11
Unconnected: 8C.7(A<B_O) 9C.7(A<B_O)

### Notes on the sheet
- Current location is A
  Endpoint is B
- Current location is A
  Endpoint is B
- Up or down? U = 0, d = 1
- Up or down? U = 0, d = 1
- MSB | MSB | (Technically right or left)
- Resets Phase Pointer

## Sheet 13 of 13: Connectors
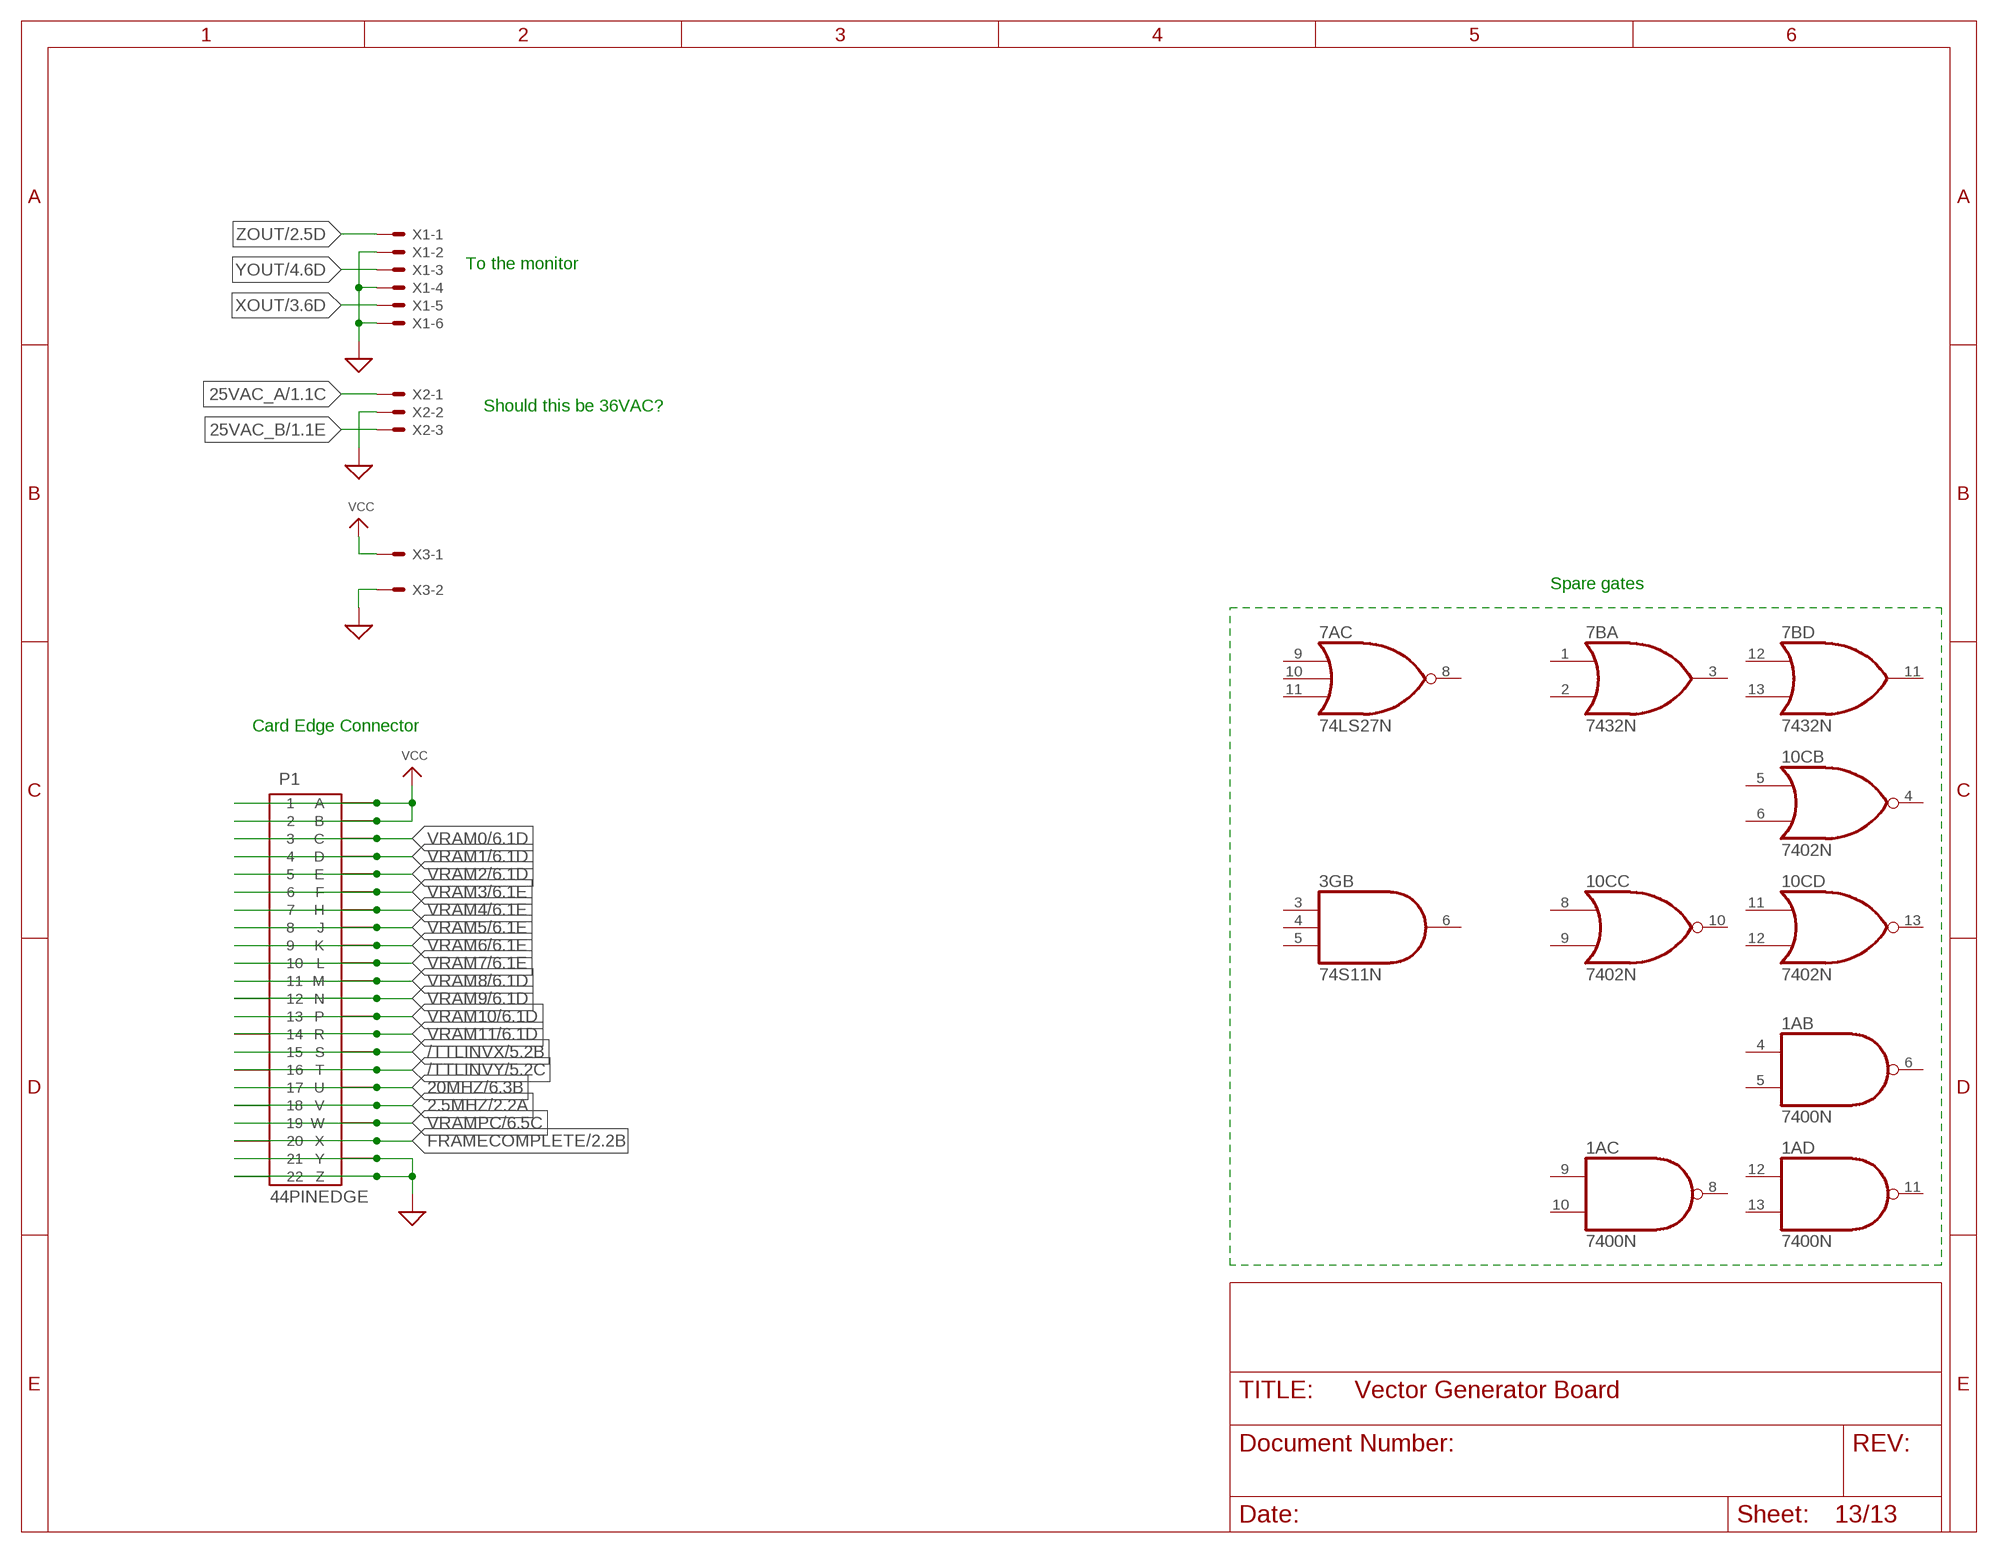
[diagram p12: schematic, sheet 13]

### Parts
P1  44PINEDGE  [44PINEDGE]
X1  KK-156-6  [KK-156-6]
X2  KK-156-3  [KK-156-3]
X3  KK-156-2  [KK-156-2]

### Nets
2.5MHZ: P1.18 P1.V ; also sheet 2,10
20MHZ: P1.17 P1.U ; also sheet 6,9
25VAC_A: X2.1 ; also sheet 1
25VAC_B: X2.3 ; also sheet 1
/TTLINVX: P1.15 P1.S ; also sheet 5
/TTLINVY: P1.16 P1.T ; also sheet 5
FRAMECOMPLETE: P1.20 P1.X ; also sheet 2,6
GND: P1.21 P1.22 P1.Y P1.Z X1.2 X1.4 X1.6 X2.2 X3.2 ; supply symbol labelled SUP ; also sheet 1,2,3,4,6,7,9,12
VCC: P1.1 P1.2 P1.A P1.B X3.1 ; also sheet 1,2
VRAM0: P1.3 P1.C ; also sheet 6
VRAM1: P1.4 P1.D ; also sheet 6
VRAM2: P1.5 P1.E ; also sheet 6
VRAM3: P1.6 P1.F ; also sheet 6
VRAM4: P1.7 P1.H ; also sheet 6
VRAM5: P1.8 P1.J ; also sheet 6
VRAM6: P1.9 P1.K ; also sheet 6
VRAM7: P1.10 P1.L ; also sheet 6
VRAM8: P1.11 P1.M ; also sheet 6
VRAM9: P1.12 P1.N ; also sheet 6
VRAM10: P1.13 P1.P ; also sheet 6
VRAM11: P1.14 P1.R ; also sheet 6
VRAMPC: P1.19 P1.W ; also sheet 6
XOUT: X1.5 ; also sheet 3
YOUT: X1.3 ; also sheet 4
ZOUT: X1.1 ; also sheet 2
Unconnected: 1A.4(B:I0) 1A.5(B:I1) 1A.6(B:O) 1A.8(C:O) 1A.9(C:I0) 1A.10(C:I1) 1A.11(D:O) 1A.12(D:I0) 1A.13(D:I1) 3G.3(B:I0) 3G.4(B:I1) 3G.5(B:I2) 3G.6(B:O) 7A.8(C:O) 7A.9(C:I0) 7A.10(C:I1) 7A.11(C:I2) 7B.1(A:I0) 7B.2(A:I1) 7B.3(A:O) 7B.11(D:O) 7B.12(D:I0) 7B.13(D:I1) 10C.4(B:O) 10C.5(B:I0) 10C.6(B:I1) 10C.8(C:I0) 10C.9(C:I1) 10C.10(C:O) 10C.11(D:I0) 10C.12(D:I1) 10C.13(D:O)

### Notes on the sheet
- To the monitor
- Should this be 36VAC?
- Spare gates
- Card Edge Connector

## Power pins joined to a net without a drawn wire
GND: 1A.7(P:GND) 1B.10(GND) 1C.10(GND) 1D.10(GND) 1E.7(P:GND) 1F.10(GND) 1G.10(GND) 1H.7(P:GND) 2A.7(P:GND) 2B.10(GND) 2C.7(P:GND) 2D.10(GND) 2E.7(P:GND) 2F.10(GND) 2G.7(P:GND) 2H.7(P:GND) 3A.12(GND) 3B.12(GND) 3C.12(GND) 3D.12(GND) 3E.12(GND) 3F.12(GND) 3G.7(P:GND) 3H.8(GND) 4A.7(GND) 4B.7(GND) 4C.7(GND) 4D.7(GND) 4E.7(GND) 4F.7(GND) 4G.7(P:GND) 4H.12(GND) 5A.8(GND) 5B.8(GND) 5C.8(GND) 5D.8(GND) 5E.8(GND) 5F.8(GND) 5G.8(GND) 5H.8(GND) 6A.8(GND) 6B.8(GND) 6C.7(P:GND) 7A.7(P:GND) 7B.7(P:GND) 7C.7(P:GND) 8A.8(GND) 8B.8(GND) 8C.8(GND) 9A.8(GND) 9B.8(GND) 9C.8(GND) 10C.7(P:GND)
VCC: 1A.14(P:VCC) 1B.20(VCC) 1C.20(VCC) 1D.20(VCC) 1E.14(P:VCC) 1F.20(VCC) 1G.20(VCC) 1H.14(P:VCC) 2A.14(P:VCC) 2B.20(VCC) 2C.14(P:VCC) 2D.20(VCC) 2E.14(P:VCC) 2F.20(VCC) 2G.14(P:VCC) 2H.14(P:VCC) 3A.5(VCC) 3B.5(VCC) 3C.5(VCC) 3D.5(VCC) 3E.5(VCC) 3F.5(VCC) 3G.14(P:VCC) 3H.16(VCC) 4A.14(VCC) 4B.14(VCC) 4C.14(VCC) 4D.14(VCC) 4E.14(VCC) 4F.14(VCC) 4G.14(P:VCC) 4H.24(VCC) 5A.16(VCC) 5B.16(VCC) 5C.16(VCC) 5D.16(VCC) 5E.16(VCC) 5F.16(VCC) 5G.16(VCC) 5H.16(VCC) 6A.16(VCC) 6B.16(VCC) 6C.14(P:VCC) 7A.14(P:VCC) 7B.14(P:VCC) 7C.14(P:VCC) 8A.16(VCC) 8B.16(VCC) 8C.16(VCC) 9A.16(VCC) 9B.16(VCC) 9C.16(VCC) 10C.14(P:VCC)

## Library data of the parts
1A = 74xx-us:74*00: Quad 2-input NAND gate
1B 1C 1D 1F 1G 2B 2D 2F = 74xx-us:74*573: 8-bit D latch BUS DRIVER
1E = 74xx-us:74*08: Quad 2-input AND gate
1H 7B = 74xx-us:74*32: Quad 2-input OR gate
2A 2C 2E 2G 2H 4G 7C = 74xx-us:74*04: Hex INVERTER
3A 3B 3C 3D 3E 3F = 74xx-us:74*83: 4-bit binary full ADDER, fast carry
3G 6C = 74xx-us:74*11: Triple 3-input AND gate
3H 5C 5D 5E 5F 5G 5H = 74xx-us:74*191: Synchronous UP/DOWN COUNTER
4A 4B 4C 4D 4E 4F = 74xx-us:74*95: 4-bit parallel access SHIFT REGISTER
4H = 74xx-us:74*154: 4-line to 16-line data SELECTOR/MULTIPLEXER
5A 5B 6A 6B = 74xx-us:74*97: Synchronous 6-bit binary rate MULTIPLIER
7A = 74xx-us:74*27: Triple 3-input NOR gate
8A 8B 8C 9A 9B 9C = 74xx-us:74*85: 4-bit magnitude COMPARATOR
10C = 74xx-us:74*02: Quad 2-input NOR gate
C1 C2 C8-C59 = rcl:C-US: CAPACITOR, American symbol; SPICEPREFIX: C
C3-C7 = rcl:CPOL-US: POLARIZED CAPACITOR, American symbol; SPICEPREFIX: C
D1-D5 = diode:1N4004: DIODE
D6 D7 = diode:ZENER-DIODE: Z-Diode
IC1-IC3 = v-reg:78XXL: VOLTAGE REGULATOR
IC7 IC12 = OLD AND OBSOLETE ARCADE PARTS:AD561
IC8 IC13 = OLD AND OBSOLETE ARCADE PARTS:DAC312: A DAC found in atari games.
IC9 IC14 = linear:TL081: OP AMP
IC10 IC15 = linear:TL082: OP AMP Data sheet; DATA_SHEET: <a href="http://www.ti.com/lit/ds/symlink/tl084a.pdf"> Data sheet </a>
IC11 IC16 = 40xx:4016: Quad bilateral ANALOG SWITCH
JP1-JP4 = pinhead:PINHD-1X12: PIN HEADER
LED1-LED4 = led:LED: LED
P1 = edge-156:44PINEDGE: 44 PIN EDGE CONNECTOR FOR PCB
Q1-Q6 = transistor-pnp:2N3906: PNP Transistor
R1-R17 R21-R24 R26 R29 R32-R36 R39 R41 R42 R45-R49 R52 R54-R66 = rcl:R-US_: RESISTOR, American symbol; SPICEPREFIX: R
R18-R20 R25 R27 R28 R30 R31 R37 R38 R40 R43 R44 R50 R51 R53 = resistor:R-US_: RESISTOR, American symbol
T1 T2 = transistor:2N3904: NPN TRANSISTOR
VR1-VR4 = SparkFun-Resistors:TRIMPOT: Trimming Potentiometer (Trimpot) Three-terminal potentiometers, with an adjustable wiper and two adjustable resistors. A pot can be used to create a configurable voltage divider, or as a variable resistor. "Trimpots" are a subset of potentiometers, usually intended for "set-and-forget"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; PROD_ID: RES-09730; SF_SKU: COM-09806
X1 = con-molex:KK-156-6: KK 156 HEADER Source: http://www.molex.com/pdm_docs/sd/026604100_sd.pdf; MF: MOLEX; OC_FARNELL: unknown; OC_NEWARK: unknown
X2 = con-molex:KK-156-3: KK 156 HEADER Source: http://www.molex.com/pdm_docs/sd/026604100_sd.pdf; MF: MOLEX; OC_FARNELL: unknown; OC_NEWARK: unknown
X3 = con-molex:KK-156-2: KK 156 HEADER; MF: MOLEX; OC_FARNELL: unknown; OC_NEWARK: unknown

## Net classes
0 default: width 0.381 mm, clearance 0.203 mm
